//   generated at:  15.06.2007 11:45:47
//   generated by:  ALPHA-VISION/DataLink2Awl
//   project:       IMAC_L
//   user:          de2zehr0

FUNCTION "abvspu_T_API_FC" : VOID
TITLE =
VERSION : 0.1


VAR_TEMP
  rVal : REAL ;
  iVal : DINT ;
  wSts : INT ;
END_VAR
BEGIN
NETWORK
TITLE =API-Testfunktionen

      AUF   "abvspu_DB_DataLinkPLC";



      CALL "GetValueI" (
           obj                      := 1, // PointId = 011010, Station = PCU1
           iVal                     := #iVal);

      L     #iVal;
      T     DBD    2;


      CALL "GetValueI" (
           obj                      := 2505, // PointId = 011080, Station = PCU1
           iVal                     := #iVal);

      L     #iVal;
      T     DBD    6;


      CALL "GetValueI" (
           obj                      := 4, // PointId = 011160, Station = PCU1
           iVal                     := #iVal);

      L     #iVal;
      T     DBD    10;


      CALL "GetValueI" (
           obj                      := 5, // PointId = 011170, Station = PCU1
           iVal                     := #iVal);

      L     #iVal;
      T     DBD    14;


      CALL "GetValueI" (
           obj                      := 6, // PointId = 011180, Station = PCU1
           iVal                     := #iVal);

      L     #iVal;
      T     DBD    18;


      CALL "GetValueI" (
           obj                      := 8, // PointId = 011200, Station = PCU1
           iVal                     := #iVal);

      L     #iVal;
      T     DBD    22;


      CALL "GetValueI" (
           obj                      := 9, // PointId = 011210, Station = PCU1
           iVal                     := #iVal);

      L     #iVal;
      T     DBD    26;


      CALL "GetValueI" (
           obj                      := 2, // PointId = 011030, Station = PCU1
           iVal                     := #iVal);

      L     #iVal;
      T     DBD    30;


      CALL "GetValueI" (
           obj                      := 7, // PointId = 011190, Station = PCU1
           iVal                     := #iVal);

      L     #iVal;
      T     DBD    34;


      CALL "GetValueI" (
           obj                      := 10, // PointId = 011570, Station = PCU1
           iVal                     := #iVal);

      L     #iVal;
      T     DBD    38;


      CALL "GetValueR" (
           obj                      := 2503, // PointId = 011060, Station = PCU1
           rVal                     := #rVal);

      L     #rVal;
      T     DBD    42;


      CALL "GetValueR" (
           obj                      := 2505, // PointId = 011080, Station = PCU1
           rVal                     := #rVal);

      L     #rVal;
      T     DBD    46;


      CALL "GetValueR" (
           obj                      := 2506, // PointId = 011090, Station = PCU1
           rVal                     := #rVal);

      L     #rVal;
      T     DBD    50;


      CALL "GetValueR" (
           obj                      := 2508, // PointId = 011110, Station = PCU1
           rVal                     := #rVal);

      L     #rVal;
      T     DBD    54;


      CALL "GetValueR" (
           obj                      := 2510, // PointId = 011130, Station = PCU1
           rVal                     := #rVal);

      L     #rVal;
      T     DBD    58;


      CALL "GetValueR" (
           obj                      := 2500, // PointId = 011020, Station = PCU1
           rVal                     := #rVal);

      L     #rVal;
      T     DBD    62;


      CALL "GetValueR" (
           obj                      := 2501, // PointId = 011040, Station = PCU1
           rVal                     := #rVal);

      L     #rVal;
      T     DBD    66;


      CALL "GetValueR" (
           obj                      := 2502, // PointId = 011050, Station = PCU1
           rVal                     := #rVal);

      L     #rVal;
      T     DBD    70;


      CALL "GetValueR" (
           obj                      := 2504, // PointId = 011070, Station = PCU1
           rVal                     := #rVal);

      L     #rVal;
      T     DBD    74;


      CALL "GetValueR" (
           obj                      := 2507, // PointId = 011100, Station = PCU1
           rVal                     := #rVal);

      L     #rVal;
      T     DBD    78;


      CALL "GetValueR" (
           obj                      := 2509, // PointId = 011120, Station = PCU1
           rVal                     := #rVal);

      L     #rVal;
      T     DBD    82;


      CALL "GetValueR" (
           obj                      := 2511, // PointId = 011140, Station = PCU1
           rVal                     := #rVal);

      L     #rVal;
      T     DBD    86;


      CALL "GetValueR" (
           obj                      := 2512, // PointId = 011230, Station = PCU1
           rVal                     := #rVal);

      L     #rVal;
      T     DBD    90;


      CALL "GetValueR" (
           obj                      := 2513, // PointId = 011240, Station = PCU1
           rVal                     := #rVal);

      L     #rVal;
      T     DBD    94;


      CALL "GetValueR" (
           obj                      := 2514, // PointId = 011250, Station = PCU1
           rVal                     := #rVal);

      L     #rVal;
      T     DBD    98;


      CALL "GetValueR" (
           obj                      := 2515, // PointId = 011260, Station = PCU1
           rVal                     := #rVal);

      L     #rVal;
      T     DBD    102;


      CALL "GetValueR" (
           obj                      := 2516, // PointId = 011270, Station = PCU1
           rVal                     := #rVal);

      L     #rVal;
      T     DBD    106;


      CALL "GetValueR" (
           obj                      := 2517, // PointId = 011280, Station = PCU1
           rVal                     := #rVal);

      L     #rVal;
      T     DBD    110;


      CALL "GetValueR" (
           obj                      := 2518, // PointId = 011290, Station = PCU1
           rVal                     := #rVal);

      L     #rVal;
      T     DBD    114;


      CALL "GetValueR" (
           obj                      := 2519, // PointId = 011300, Station = PCU1
           rVal                     := #rVal);

      L     #rVal;
      T     DBD    118;


      CALL "GetValueR" (
           obj                      := 2520, // PointId = 011310, Station = PCU1
           rVal                     := #rVal);

      L     #rVal;
      T     DBD    122;


      CALL "GetValueR" (
           obj                      := 2521, // PointId = 011320, Station = PCU1
           rVal                     := #rVal);

      L     #rVal;
      T     DBD    126;


      CALL "GetValueR" (
           obj                      := 2522, // PointId = 011330, Station = PCU1
           rVal                     := #rVal);

      L     #rVal;
      T     DBD    130;


      CALL "GetValueR" (
           obj                      := 2523, // PointId = 011340, Station = PCU1
           rVal                     := #rVal);

      L     #rVal;
      T     DBD    134;


      CALL "GetValueR" (
           obj                      := 2524, // PointId = 011350, Station = PCU1
           rVal                     := #rVal);

      L     #rVal;
      T     DBD    138;


      CALL "GetValueR" (
           obj                      := 2525, // PointId = 011360, Station = PCU1
           rVal                     := #rVal);

      L     #rVal;
      T     DBD    142;


      CALL "GetValueR" (
           obj                      := 2526, // PointId = 011370, Station = PCU1
           rVal                     := #rVal);

      L     #rVal;
      T     DBD    146;


      CALL "GetValueR" (
           obj                      := 2527, // PointId = 011380, Station = PCU1
           rVal                     := #rVal);

      L     #rVal;
      T     DBD    150;


      CALL "GetValueR" (
           obj                      := 2544, // PointId = 011550, Station = PCU1
           rVal                     := #rVal);

      L     #rVal;
      T     DBD    154;


      CALL "GetValueR" (
           obj                      := 2545, // PointId = 011560, Station = PCU1
           rVal                     := #rVal);

      L     #rVal;
      T     DBD    158;


      CALL "GetValueI" (
           obj                      := 13, // PointId = 012010, Station = PCU1
           iVal                     := #iVal);

      L     #iVal;
      T     DBD    162;


      CALL "GetValueI" (
           obj                      := 2551, // PointId = 012080, Station = PCU1
           iVal                     := #iVal);

      L     #iVal;
      T     DBD    166;


      CALL "GetValueI" (
           obj                      := 16, // PointId = 012160, Station = PCU1
           iVal                     := #iVal);

      L     #iVal;
      T     DBD    170;


      CALL "GetValueI" (
           obj                      := 17, // PointId = 012170, Station = PCU1
           iVal                     := #iVal);

      L     #iVal;
      T     DBD    174;


      CALL "GetValueI" (
           obj                      := 18, // PointId = 012180, Station = PCU1
           iVal                     := #iVal);

      L     #iVal;
      T     DBD    178;


      CALL "GetValueI" (
           obj                      := 20, // PointId = 012200, Station = PCU1
           iVal                     := #iVal);

      L     #iVal;
      T     DBD    182;


      CALL "GetValueI" (
           obj                      := 21, // PointId = 012210, Station = PCU1
           iVal                     := #iVal);

      L     #iVal;
      T     DBD    186;


      CALL "GetValueI" (
           obj                      := 14, // PointId = 012030, Station = PCU1
           iVal                     := #iVal);

      L     #iVal;
      T     DBD    190;


      CALL "GetValueI" (
           obj                      := 19, // PointId = 012190, Station = PCU1
           iVal                     := #iVal);

      L     #iVal;
      T     DBD    194;


      CALL "GetValueI" (
           obj                      := 22, // PointId = 012570, Station = PCU1
           iVal                     := #iVal);

      L     #iVal;
      T     DBD    198;


      CALL "GetValueR" (
           obj                      := 2549, // PointId = 012060, Station = PCU1
           rVal                     := #rVal);

      L     #rVal;
      T     DBD    202;


      CALL "GetValueR" (
           obj                      := 2551, // PointId = 012080, Station = PCU1
           rVal                     := #rVal);

      L     #rVal;
      T     DBD    206;


      CALL "GetValueR" (
           obj                      := 2552, // PointId = 012090, Station = PCU1
           rVal                     := #rVal);

      L     #rVal;
      T     DBD    210;


      CALL "GetValueR" (
           obj                      := 2554, // PointId = 012110, Station = PCU1
           rVal                     := #rVal);

      L     #rVal;
      T     DBD    214;


      CALL "GetValueR" (
           obj                      := 2556, // PointId = 012130, Station = PCU1
           rVal                     := #rVal);

      L     #rVal;
      T     DBD    218;


      CALL "GetValueR" (
           obj                      := 2546, // PointId = 012020, Station = PCU1
           rVal                     := #rVal);

      L     #rVal;
      T     DBD    222;


      CALL "GetValueR" (
           obj                      := 2547, // PointId = 012040, Station = PCU1
           rVal                     := #rVal);

      L     #rVal;
      T     DBD    226;


      CALL "GetValueR" (
           obj                      := 2548, // PointId = 012050, Station = PCU1
           rVal                     := #rVal);

      L     #rVal;
      T     DBD    230;


      CALL "GetValueR" (
           obj                      := 2550, // PointId = 012070, Station = PCU1
           rVal                     := #rVal);

      L     #rVal;
      T     DBD    234;


      CALL "GetValueR" (
           obj                      := 2553, // PointId = 012100, Station = PCU1
           rVal                     := #rVal);

      L     #rVal;
      T     DBD    238;


      CALL "GetValueR" (
           obj                      := 2555, // PointId = 012120, Station = PCU1
           rVal                     := #rVal);

      L     #rVal;
      T     DBD    242;


      CALL "GetValueR" (
           obj                      := 2557, // PointId = 012140, Station = PCU1
           rVal                     := #rVal);

      L     #rVal;
      T     DBD    246;


      CALL "GetValueR" (
           obj                      := 2558, // PointId = 012230, Station = PCU1
           rVal                     := #rVal);

      L     #rVal;
      T     DBD    250;


      CALL "GetValueR" (
           obj                      := 2559, // PointId = 012240, Station = PCU1
           rVal                     := #rVal);

      L     #rVal;
      T     DBD    254;


      CALL "GetValueR" (
           obj                      := 2560, // PointId = 012250, Station = PCU1
           rVal                     := #rVal);

      L     #rVal;
      T     DBD    258;


      CALL "GetValueR" (
           obj                      := 2561, // PointId = 012260, Station = PCU1
           rVal                     := #rVal);

      L     #rVal;
      T     DBD    262;


      CALL "GetValueR" (
           obj                      := 2562, // PointId = 012270, Station = PCU1
           rVal                     := #rVal);

      L     #rVal;
      T     DBD    266;


      CALL "GetValueR" (
           obj                      := 2563, // PointId = 012280, Station = PCU1
           rVal                     := #rVal);

      L     #rVal;
      T     DBD    270;


      CALL "GetValueR" (
           obj                      := 2564, // PointId = 012290, Station = PCU1
           rVal                     := #rVal);

      L     #rVal;
      T     DBD    274;


      CALL "GetValueR" (
           obj                      := 2565, // PointId = 012300, Station = PCU1
           rVal                     := #rVal);

      L     #rVal;
      T     DBD    278;


      CALL "GetValueR" (
           obj                      := 2566, // PointId = 012310, Station = PCU1
           rVal                     := #rVal);

      L     #rVal;
      T     DBD    282;


      CALL "GetValueR" (
           obj                      := 2567, // PointId = 012320, Station = PCU1
           rVal                     := #rVal);

      L     #rVal;
      T     DBD    286;


      CALL "GetValueR" (
           obj                      := 2568, // PointId = 012330, Station = PCU1
           rVal                     := #rVal);

      L     #rVal;
      T     DBD    290;


      CALL "GetValueR" (
           obj                      := 2569, // PointId = 012340, Station = PCU1
           rVal                     := #rVal);

      L     #rVal;
      T     DBD    294;


      CALL "GetValueR" (
           obj                      := 2570, // PointId = 012350, Station = PCU1
           rVal                     := #rVal);

      L     #rVal;
      T     DBD    298;


      CALL "GetValueR" (
           obj                      := 2571, // PointId = 012360, Station = PCU1
           rVal                     := #rVal);

      L     #rVal;
      T     DBD    302;


      CALL "GetValueR" (
           obj                      := 2572, // PointId = 012370, Station = PCU1
           rVal                     := #rVal);

      L     #rVal;
      T     DBD    306;


      CALL "GetValueR" (
           obj                      := 2573, // PointId = 012380, Station = PCU1
           rVal                     := #rVal);

      L     #rVal;
      T     DBD    310;


      CALL "GetValueR" (
           obj                      := 2590, // PointId = 012550, Station = PCU1
           rVal                     := #rVal);

      L     #rVal;
      T     DBD    314;


      CALL "GetValueR" (
           obj                      := 2591, // PointId = 012560, Station = PCU1
           rVal                     := #rVal);

      L     #rVal;
      T     DBD    318;


      CALL "GetValueR" (
           obj                      := 2883, // PointId = 021010, Station = PCU1
           rVal                     := #rVal);

      L     #rVal;
      T     DBD    322;


      CALL "GetValueR" (
           obj                      := 2884, // PointId = 021020, Station = PCU1
           rVal                     := #rVal);

      L     #rVal;
      T     DBD    326;


      CALL "GetValueR" (
           obj                      := 2885, // PointId = 021030, Station = PCU1
           rVal                     := #rVal);

      L     #rVal;
      T     DBD    330;


      CALL "GetValueR" (
           obj                      := 2886, // PointId = 021040, Station = PCU1
           rVal                     := #rVal);

      L     #rVal;
      T     DBD    334;


      CALL "GetValueR" (
           obj                      := 2887, // PointId = 021051, Station = PCU1
           rVal                     := #rVal);

      L     #rVal;
      T     DBD    338;


      CALL "GetValueR" (
           obj                      := 2888, // PointId = 021060, Station = PCU1
           rVal                     := #rVal);

      L     #rVal;
      T     DBD    342;


      CALL "GetValueR" (
           obj                      := 2889, // PointId = 021070, Station = PCU1
           rVal                     := #rVal);

      L     #rVal;
      T     DBD    346;


      CALL "GetValueR" (
           obj                      := 2890, // PointId = 021080, Station = PCU1
           rVal                     := #rVal);

      L     #rVal;
      T     DBD    350;


      CALL "GetValueR" (
           obj                      := 2891, // PointId = 021090, Station = PCU1
           rVal                     := #rVal);

      L     #rVal;
      T     DBD    354;


      CALL "GetValueR" (
           obj                      := 2892, // PointId = 021120, Station = PCU1
           rVal                     := #rVal);

      L     #rVal;
      T     DBD    358;


      CALL "GetValueR" (
           obj                      := 2893, // PointId = 021130, Station = PCU1
           rVal                     := #rVal);

      L     #rVal;
      T     DBD    362;


      CALL "GetValueR" (
           obj                      := 2894, // PointId = 021140, Station = PCU1
           rVal                     := #rVal);

      L     #rVal;
      T     DBD    366;


      CALL "GetValueR" (
           obj                      := 2895, // PointId = 021150, Station = PCU1
           rVal                     := #rVal);

      L     #rVal;
      T     DBD    370;


      CALL "GetValueR" (
           obj                      := 2896, // PointId = 021160, Station = PCU1
           rVal                     := #rVal);

      L     #rVal;
      T     DBD    374;


      CALL "GetValueR" (
           obj                      := 2897, // PointId = 021170, Station = PCU1
           rVal                     := #rVal);

      L     #rVal;
      T     DBD    378;


      CALL "GetValueR" (
           obj                      := 2898, // PointId = 021180, Station = PCU1
           rVal                     := #rVal);

      L     #rVal;
      T     DBD    382;


      CALL "GetValueI" (
           obj                      := 140, // PointId = 021100, Station = PCU1
           iVal                     := #iVal);

      L     #iVal;
      T     DBD    386;


      CALL "GetValueI" (
           obj                      := 141, // PointId = 021110, Station = PCU1
           iVal                     := #iVal);

      L     #iVal;
      T     DBD    390;


      CALL "GetValueI" (
           obj                      := 142, // PointId = 021190, Station = PCU1
           iVal                     := #iVal);

      L     #iVal;
      T     DBD    394;


      CALL "GetValueI" (
           obj                      := 143, // PointId = 021200, Station = PCU1
           iVal                     := #iVal);

      L     #iVal;
      T     DBD    398;


      CALL "GetValueI" (
           obj                      := 144, // PointId = 021210, Station = PCU1
           iVal                     := #iVal);

      L     #iVal;
      T     DBD    402;


      CALL "GetValueI" (
           obj                      := 145, // PointId = 021240, Station = PCU1
           iVal                     := #iVal);

      L     #iVal;
      T     DBD    406;


      CALL "GetValueI" (
           obj                      := 146, // PointId = 021260, Station = PCU1
           iVal                     := #iVal);

      L     #iVal;
      T     DBD    410;


      CALL "GetValueI" (
           obj                      := 147, // PointId = 021270, Station = PCU1
           iVal                     := #iVal);

      L     #iVal;
      T     DBD    414;


      CALL "GetValueI" (
           obj                      := 148, // PointId = 021290, Station = PCU1
           iVal                     := #iVal);

      L     #iVal;
      T     DBD    418;


      CALL "GetValueI" (
           obj                      := 149, // PointId = 021310, Station = PCU1
           iVal                     := #iVal);

      L     #iVal;
      T     DBD    422;


      CALL "GetValueR" (
           obj                      := 2900, // PointId = 021300, Station = PCU1
           rVal                     := #rVal);

      L     #rVal;
      T     DBD    426;


      CALL "GetValueR" (
           obj                      := 2901, // PointId = 022010, Station = PCU1
           rVal                     := #rVal);

      L     #rVal;
      T     DBD    430;


      CALL "GetValueR" (
           obj                      := 2902, // PointId = 022020, Station = PCU1
           rVal                     := #rVal);

      L     #rVal;
      T     DBD    434;


      CALL "GetValueR" (
           obj                      := 2903, // PointId = 022030, Station = PCU1
           rVal                     := #rVal);

      L     #rVal;
      T     DBD    438;


      CALL "GetValueR" (
           obj                      := 2904, // PointId = 022040, Station = PCU1
           rVal                     := #rVal);

      L     #rVal;
      T     DBD    442;


      CALL "GetValueR" (
           obj                      := 2905, // PointId = 022051, Station = PCU1
           rVal                     := #rVal);

      L     #rVal;
      T     DBD    446;


      CALL "GetValueR" (
           obj                      := 2906, // PointId = 022060, Station = PCU1
           rVal                     := #rVal);

      L     #rVal;
      T     DBD    450;


      CALL "GetValueR" (
           obj                      := 2907, // PointId = 022070, Station = PCU1
           rVal                     := #rVal);

      L     #rVal;
      T     DBD    454;


      CALL "GetValueR" (
           obj                      := 2908, // PointId = 022080, Station = PCU1
           rVal                     := #rVal);

      L     #rVal;
      T     DBD    458;


      CALL "GetValueR" (
           obj                      := 2909, // PointId = 022090, Station = PCU1
           rVal                     := #rVal);

      L     #rVal;
      T     DBD    462;


      CALL "GetValueR" (
           obj                      := 2910, // PointId = 022120, Station = PCU1
           rVal                     := #rVal);

      L     #rVal;
      T     DBD    466;


      CALL "GetValueR" (
           obj                      := 2911, // PointId = 022130, Station = PCU1
           rVal                     := #rVal);

      L     #rVal;
      T     DBD    470;


      CALL "GetValueR" (
           obj                      := 2912, // PointId = 022140, Station = PCU1
           rVal                     := #rVal);

      L     #rVal;
      T     DBD    474;


      CALL "GetValueR" (
           obj                      := 2913, // PointId = 022150, Station = PCU1
           rVal                     := #rVal);

      L     #rVal;
      T     DBD    478;


      CALL "GetValueR" (
           obj                      := 2914, // PointId = 022160, Station = PCU1
           rVal                     := #rVal);

      L     #rVal;
      T     DBD    482;


      CALL "GetValueR" (
           obj                      := 2915, // PointId = 022170, Station = PCU1
           rVal                     := #rVal);

      L     #rVal;
      T     DBD    486;


      CALL "GetValueR" (
           obj                      := 2916, // PointId = 022180, Station = PCU1
           rVal                     := #rVal);

      L     #rVal;
      T     DBD    490;


      CALL "GetValueI" (
           obj                      := 152, // PointId = 022100, Station = PCU1
           iVal                     := #iVal);

      L     #iVal;
      T     DBD    494;


      CALL "GetValueI" (
           obj                      := 153, // PointId = 022110, Station = PCU1
           iVal                     := #iVal);

      L     #iVal;
      T     DBD    498;


      CALL "GetValueI" (
           obj                      := 154, // PointId = 022190, Station = PCU1
           iVal                     := #iVal);

      L     #iVal;
      T     DBD    502;


      CALL "GetValueI" (
           obj                      := 155, // PointId = 022200, Station = PCU1
           iVal                     := #iVal);

      L     #iVal;
      T     DBD    506;


      CALL "GetValueI" (
           obj                      := 156, // PointId = 022210, Station = PCU1
           iVal                     := #iVal);

      L     #iVal;
      T     DBD    510;


      CALL "GetValueI" (
           obj                      := 157, // PointId = 022240, Station = PCU1
           iVal                     := #iVal);

      L     #iVal;
      T     DBD    514;


      CALL "GetValueI" (
           obj                      := 158, // PointId = 022260, Station = PCU1
           iVal                     := #iVal);

      L     #iVal;
      T     DBD    518;


      CALL "GetValueI" (
           obj                      := 159, // PointId = 022270, Station = PCU1
           iVal                     := #iVal);

      L     #iVal;
      T     DBD    522;


      CALL "GetValueI" (
           obj                      := 160, // PointId = 022290, Station = PCU1
           iVal                     := #iVal);

      L     #iVal;
      T     DBD    526;


      CALL "GetValueI" (
           obj                      := 161, // PointId = 022310, Station = PCU1
           iVal                     := #iVal);

      L     #iVal;
      T     DBD    530;


      CALL "GetValueR" (
           obj                      := 2918, // PointId = 022300, Station = PCU1
           rVal                     := #rVal);

      L     #rVal;
      T     DBD    534;


      CALL "GetValueI" (
           obj                      := 25, // PointId = 013010, Station = PCU1
           iVal                     := #iVal);

      L     #iVal;
      T     DBD    538;


      CALL "GetValueI" (
           obj                      := 2597, // PointId = 013080, Station = PCU1
           iVal                     := #iVal);

      L     #iVal;
      T     DBD    542;


      CALL "GetValueI" (
           obj                      := 28, // PointId = 013160, Station = PCU1
           iVal                     := #iVal);

      L     #iVal;
      T     DBD    546;


      CALL "GetValueI" (
           obj                      := 29, // PointId = 013170, Station = PCU1
           iVal                     := #iVal);

      L     #iVal;
      T     DBD    550;


      CALL "GetValueI" (
           obj                      := 30, // PointId = 013180, Station = PCU1
           iVal                     := #iVal);

      L     #iVal;
      T     DBD    554;


      CALL "GetValueI" (
           obj                      := 32, // PointId = 013200, Station = PCU1
           iVal                     := #iVal);

      L     #iVal;
      T     DBD    558;


      CALL "GetValueI" (
           obj                      := 33, // PointId = 013210, Station = PCU1
           iVal                     := #iVal);

      L     #iVal;
      T     DBD    562;


      CALL "GetValueI" (
           obj                      := 26, // PointId = 013030, Station = PCU1
           iVal                     := #iVal);

      L     #iVal;
      T     DBD    566;


      CALL "GetValueI" (
           obj                      := 31, // PointId = 013190, Station = PCU1
           iVal                     := #iVal);

      L     #iVal;
      T     DBD    570;


      CALL "GetValueI" (
           obj                      := 34, // PointId = 013570, Station = PCU1
           iVal                     := #iVal);

      L     #iVal;
      T     DBD    574;


      CALL "GetValueR" (
           obj                      := 2595, // PointId = 013060, Station = PCU1
           rVal                     := #rVal);

      L     #rVal;
      T     DBD    578;


      CALL "GetValueR" (
           obj                      := 2597, // PointId = 013080, Station = PCU1
           rVal                     := #rVal);

      L     #rVal;
      T     DBD    582;


      CALL "GetValueR" (
           obj                      := 2598, // PointId = 013090, Station = PCU1
           rVal                     := #rVal);

      L     #rVal;
      T     DBD    586;


      CALL "GetValueR" (
           obj                      := 2600, // PointId = 013110, Station = PCU1
           rVal                     := #rVal);

      L     #rVal;
      T     DBD    590;


      CALL "GetValueR" (
           obj                      := 2602, // PointId = 013130, Station = PCU1
           rVal                     := #rVal);

      L     #rVal;
      T     DBD    594;


      CALL "GetValueR" (
           obj                      := 2592, // PointId = 013020, Station = PCU1
           rVal                     := #rVal);

      L     #rVal;
      T     DBD    598;


      CALL "GetValueR" (
           obj                      := 2593, // PointId = 013040, Station = PCU1
           rVal                     := #rVal);

      L     #rVal;
      T     DBD    602;


      CALL "GetValueR" (
           obj                      := 2594, // PointId = 013050, Station = PCU1
           rVal                     := #rVal);

      L     #rVal;
      T     DBD    606;


      CALL "GetValueR" (
           obj                      := 2596, // PointId = 013070, Station = PCU1
           rVal                     := #rVal);

      L     #rVal;
      T     DBD    610;


      CALL "GetValueR" (
           obj                      := 2599, // PointId = 013100, Station = PCU1
           rVal                     := #rVal);

      L     #rVal;
      T     DBD    614;


      CALL "GetValueR" (
           obj                      := 2601, // PointId = 013120, Station = PCU1
           rVal                     := #rVal);

      L     #rVal;
      T     DBD    618;


      CALL "GetValueR" (
           obj                      := 2603, // PointId = 013140, Station = PCU1
           rVal                     := #rVal);

      L     #rVal;
      T     DBD    622;


      CALL "GetValueR" (
           obj                      := 2604, // PointId = 013230, Station = PCU1
           rVal                     := #rVal);

      L     #rVal;
      T     DBD    626;


      CALL "GetValueR" (
           obj                      := 2605, // PointId = 013240, Station = PCU1
           rVal                     := #rVal);

      L     #rVal;
      T     DBD    630;


      CALL "GetValueR" (
           obj                      := 2606, // PointId = 013250, Station = PCU1
           rVal                     := #rVal);

      L     #rVal;
      T     DBD    634;


      CALL "GetValueR" (
           obj                      := 2607, // PointId = 013260, Station = PCU1
           rVal                     := #rVal);

      L     #rVal;
      T     DBD    638;


      CALL "GetValueR" (
           obj                      := 2608, // PointId = 013270, Station = PCU1
           rVal                     := #rVal);

      L     #rVal;
      T     DBD    642;


      CALL "GetValueR" (
           obj                      := 2609, // PointId = 013280, Station = PCU1
           rVal                     := #rVal);

      L     #rVal;
      T     DBD    646;


      CALL "GetValueR" (
           obj                      := 2610, // PointId = 013290, Station = PCU1
           rVal                     := #rVal);

      L     #rVal;
      T     DBD    650;


      CALL "GetValueR" (
           obj                      := 2611, // PointId = 013300, Station = PCU1
           rVal                     := #rVal);

      L     #rVal;
      T     DBD    654;


      CALL "GetValueR" (
           obj                      := 2612, // PointId = 013310, Station = PCU1
           rVal                     := #rVal);

      L     #rVal;
      T     DBD    658;


      CALL "GetValueR" (
           obj                      := 2613, // PointId = 013320, Station = PCU1
           rVal                     := #rVal);

      L     #rVal;
      T     DBD    662;


      CALL "GetValueR" (
           obj                      := 2614, // PointId = 013330, Station = PCU1
           rVal                     := #rVal);

      L     #rVal;
      T     DBD    666;


      CALL "GetValueR" (
           obj                      := 2615, // PointId = 013340, Station = PCU1
           rVal                     := #rVal);

      L     #rVal;
      T     DBD    670;


      CALL "GetValueR" (
           obj                      := 2616, // PointId = 013350, Station = PCU1
           rVal                     := #rVal);

      L     #rVal;
      T     DBD    674;


      CALL "GetValueR" (
           obj                      := 2617, // PointId = 013360, Station = PCU1
           rVal                     := #rVal);

      L     #rVal;
      T     DBD    678;


      CALL "GetValueR" (
           obj                      := 2618, // PointId = 013370, Station = PCU1
           rVal                     := #rVal);

      L     #rVal;
      T     DBD    682;


      CALL "GetValueR" (
           obj                      := 2619, // PointId = 013380, Station = PCU1
           rVal                     := #rVal);

      L     #rVal;
      T     DBD    686;


      CALL "GetValueR" (
           obj                      := 2636, // PointId = 013550, Station = PCU1
           rVal                     := #rVal);

      L     #rVal;
      T     DBD    690;


      CALL "GetValueR" (
           obj                      := 2637, // PointId = 013560, Station = PCU1
           rVal                     := #rVal);

      L     #rVal;
      T     DBD    694;


      CALL "GetValueI" (
           obj                      := 37, // PointId = 014010, Station = PCU1
           iVal                     := #iVal);

      L     #iVal;
      T     DBD    698;


      CALL "GetValueI" (
           obj                      := 2643, // PointId = 014080, Station = PCU1
           iVal                     := #iVal);

      L     #iVal;
      T     DBD    702;


      CALL "GetValueI" (
           obj                      := 40, // PointId = 014160, Station = PCU1
           iVal                     := #iVal);

      L     #iVal;
      T     DBD    706;


      CALL "GetValueI" (
           obj                      := 41, // PointId = 014170, Station = PCU1
           iVal                     := #iVal);

      L     #iVal;
      T     DBD    710;


      CALL "GetValueI" (
           obj                      := 42, // PointId = 014180, Station = PCU1
           iVal                     := #iVal);

      L     #iVal;
      T     DBD    714;


      CALL "GetValueI" (
           obj                      := 44, // PointId = 014200, Station = PCU1
           iVal                     := #iVal);

      L     #iVal;
      T     DBD    718;


      CALL "GetValueI" (
           obj                      := 45, // PointId = 014210, Station = PCU1
           iVal                     := #iVal);

      L     #iVal;
      T     DBD    722;


      CALL "GetValueI" (
           obj                      := 38, // PointId = 014030, Station = PCU1
           iVal                     := #iVal);

      L     #iVal;
      T     DBD    726;


      CALL "GetValueI" (
           obj                      := 43, // PointId = 014190, Station = PCU1
           iVal                     := #iVal);

      L     #iVal;
      T     DBD    730;


      CALL "GetValueI" (
           obj                      := 46, // PointId = 014570, Station = PCU1
           iVal                     := #iVal);

      L     #iVal;
      T     DBD    734;


      CALL "GetValueR" (
           obj                      := 2641, // PointId = 014060, Station = PCU1
           rVal                     := #rVal);

      L     #rVal;
      T     DBD    738;


      CALL "GetValueR" (
           obj                      := 2643, // PointId = 014080, Station = PCU1
           rVal                     := #rVal);

      L     #rVal;
      T     DBD    742;


      CALL "GetValueR" (
           obj                      := 2644, // PointId = 014090, Station = PCU1
           rVal                     := #rVal);

      L     #rVal;
      T     DBD    746;


      CALL "GetValueR" (
           obj                      := 2646, // PointId = 014110, Station = PCU1
           rVal                     := #rVal);

      L     #rVal;
      T     DBD    750;


      CALL "GetValueR" (
           obj                      := 2648, // PointId = 014130, Station = PCU1
           rVal                     := #rVal);

      L     #rVal;
      T     DBD    754;


      CALL "GetValueR" (
           obj                      := 2638, // PointId = 014020, Station = PCU1
           rVal                     := #rVal);

      L     #rVal;
      T     DBD    758;


      CALL "GetValueR" (
           obj                      := 2639, // PointId = 014040, Station = PCU1
           rVal                     := #rVal);

      L     #rVal;
      T     DBD    762;


      CALL "GetValueR" (
           obj                      := 2640, // PointId = 014050, Station = PCU1
           rVal                     := #rVal);

      L     #rVal;
      T     DBD    766;


      CALL "GetValueR" (
           obj                      := 2642, // PointId = 014070, Station = PCU1
           rVal                     := #rVal);

      L     #rVal;
      T     DBD    770;


      CALL "GetValueR" (
           obj                      := 2645, // PointId = 014100, Station = PCU1
           rVal                     := #rVal);

      L     #rVal;
      T     DBD    774;


      CALL "GetValueR" (
           obj                      := 2647, // PointId = 014120, Station = PCU1
           rVal                     := #rVal);

      L     #rVal;
      T     DBD    778;


      CALL "GetValueR" (
           obj                      := 2649, // PointId = 014140, Station = PCU1
           rVal                     := #rVal);

      L     #rVal;
      T     DBD    782;


      CALL "GetValueR" (
           obj                      := 2650, // PointId = 014230, Station = PCU1
           rVal                     := #rVal);

      L     #rVal;
      T     DBD    786;


      CALL "GetValueR" (
           obj                      := 2651, // PointId = 014240, Station = PCU1
           rVal                     := #rVal);

      L     #rVal;
      T     DBD    790;


      CALL "GetValueR" (
           obj                      := 2652, // PointId = 014250, Station = PCU1
           rVal                     := #rVal);

      L     #rVal;
      T     DBD    794;


      CALL "GetValueR" (
           obj                      := 2653, // PointId = 014260, Station = PCU1
           rVal                     := #rVal);

      L     #rVal;
      T     DBD    798;


      CALL "GetValueR" (
           obj                      := 2654, // PointId = 014270, Station = PCU1
           rVal                     := #rVal);

      L     #rVal;
      T     DBD    802;


      CALL "GetValueR" (
           obj                      := 2655, // PointId = 014280, Station = PCU1
           rVal                     := #rVal);

      L     #rVal;
      T     DBD    806;


      CALL "GetValueR" (
           obj                      := 2656, // PointId = 014290, Station = PCU1
           rVal                     := #rVal);

      L     #rVal;
      T     DBD    810;


      CALL "GetValueR" (
           obj                      := 2657, // PointId = 014300, Station = PCU1
           rVal                     := #rVal);

      L     #rVal;
      T     DBD    814;


      CALL "GetValueR" (
           obj                      := 2658, // PointId = 014310, Station = PCU1
           rVal                     := #rVal);

      L     #rVal;
      T     DBD    818;


      CALL "GetValueR" (
           obj                      := 2659, // PointId = 014320, Station = PCU1
           rVal                     := #rVal);

      L     #rVal;
      T     DBD    822;


      CALL "GetValueR" (
           obj                      := 2660, // PointId = 014330, Station = PCU1
           rVal                     := #rVal);

      L     #rVal;
      T     DBD    826;


      CALL "GetValueR" (
           obj                      := 2661, // PointId = 014340, Station = PCU1
           rVal                     := #rVal);

      L     #rVal;
      T     DBD    830;


      CALL "GetValueR" (
           obj                      := 2662, // PointId = 014350, Station = PCU1
           rVal                     := #rVal);

      L     #rVal;
      T     DBD    834;


      CALL "GetValueR" (
           obj                      := 2663, // PointId = 014360, Station = PCU1
           rVal                     := #rVal);

      L     #rVal;
      T     DBD    838;


      CALL "GetValueR" (
           obj                      := 2664, // PointId = 014370, Station = PCU1
           rVal                     := #rVal);

      L     #rVal;
      T     DBD    842;


      CALL "GetValueR" (
           obj                      := 2665, // PointId = 014380, Station = PCU1
           rVal                     := #rVal);

      L     #rVal;
      T     DBD    846;


      CALL "GetValueR" (
           obj                      := 2682, // PointId = 014550, Station = PCU1
           rVal                     := #rVal);

      L     #rVal;
      T     DBD    850;


      CALL "GetValueR" (
           obj                      := 2683, // PointId = 014560, Station = PCU1
           rVal                     := #rVal);

      L     #rVal;
      T     DBD    854;


      CALL "GetValueR" (
           obj                      := 2919, // PointId = 023010, Station = PCU1
           rVal                     := #rVal);

      L     #rVal;
      T     DBD    858;


      CALL "GetValueR" (
           obj                      := 2920, // PointId = 023020, Station = PCU1
           rVal                     := #rVal);

      L     #rVal;
      T     DBD    862;


      CALL "GetValueR" (
           obj                      := 2921, // PointId = 023030, Station = PCU1
           rVal                     := #rVal);

      L     #rVal;
      T     DBD    866;


      CALL "GetValueR" (
           obj                      := 2922, // PointId = 023040, Station = PCU1
           rVal                     := #rVal);

      L     #rVal;
      T     DBD    870;


      CALL "GetValueR" (
           obj                      := 2923, // PointId = 023051, Station = PCU1
           rVal                     := #rVal);

      L     #rVal;
      T     DBD    874;


      CALL "GetValueR" (
           obj                      := 2924, // PointId = 023060, Station = PCU1
           rVal                     := #rVal);

      L     #rVal;
      T     DBD    878;


      CALL "GetValueR" (
           obj                      := 2925, // PointId = 023070, Station = PCU1
           rVal                     := #rVal);

      L     #rVal;
      T     DBD    882;


      CALL "GetValueR" (
           obj                      := 2926, // PointId = 023080, Station = PCU1
           rVal                     := #rVal);

      L     #rVal;
      T     DBD    886;


      CALL "GetValueR" (
           obj                      := 2927, // PointId = 023090, Station = PCU1
           rVal                     := #rVal);

      L     #rVal;
      T     DBD    890;


      CALL "GetValueR" (
           obj                      := 2928, // PointId = 023120, Station = PCU1
           rVal                     := #rVal);

      L     #rVal;
      T     DBD    894;


      CALL "GetValueR" (
           obj                      := 2929, // PointId = 023130, Station = PCU1
           rVal                     := #rVal);

      L     #rVal;
      T     DBD    898;


      CALL "GetValueR" (
           obj                      := 2930, // PointId = 023140, Station = PCU1
           rVal                     := #rVal);

      L     #rVal;
      T     DBD    902;


      CALL "GetValueR" (
           obj                      := 2931, // PointId = 023150, Station = PCU1
           rVal                     := #rVal);

      L     #rVal;
      T     DBD    906;


      CALL "GetValueR" (
           obj                      := 2932, // PointId = 023160, Station = PCU1
           rVal                     := #rVal);

      L     #rVal;
      T     DBD    910;


      CALL "GetValueR" (
           obj                      := 2933, // PointId = 023170, Station = PCU1
           rVal                     := #rVal);

      L     #rVal;
      T     DBD    914;


      CALL "GetValueR" (
           obj                      := 2934, // PointId = 023180, Station = PCU1
           rVal                     := #rVal);

      L     #rVal;
      T     DBD    918;


      CALL "GetValueI" (
           obj                      := 164, // PointId = 023100, Station = PCU1
           iVal                     := #iVal);

      L     #iVal;
      T     DBD    922;


      CALL "GetValueI" (
           obj                      := 165, // PointId = 023110, Station = PCU1
           iVal                     := #iVal);

      L     #iVal;
      T     DBD    926;


      CALL "GetValueI" (
           obj                      := 166, // PointId = 023190, Station = PCU1
           iVal                     := #iVal);

      L     #iVal;
      T     DBD    930;


      CALL "GetValueI" (
           obj                      := 167, // PointId = 023200, Station = PCU1
           iVal                     := #iVal);

      L     #iVal;
      T     DBD    934;


      CALL "GetValueI" (
           obj                      := 168, // PointId = 023210, Station = PCU1
           iVal                     := #iVal);

      L     #iVal;
      T     DBD    938;


      CALL "GetValueI" (
           obj                      := 169, // PointId = 023240, Station = PCU1
           iVal                     := #iVal);

      L     #iVal;
      T     DBD    942;


      CALL "GetValueI" (
           obj                      := 170, // PointId = 023260, Station = PCU1
           iVal                     := #iVal);

      L     #iVal;
      T     DBD    946;


      CALL "GetValueI" (
           obj                      := 171, // PointId = 023270, Station = PCU1
           iVal                     := #iVal);

      L     #iVal;
      T     DBD    950;


      CALL "GetValueI" (
           obj                      := 172, // PointId = 023290, Station = PCU1
           iVal                     := #iVal);

      L     #iVal;
      T     DBD    954;


      CALL "GetValueI" (
           obj                      := 173, // PointId = 023310, Station = PCU1
           iVal                     := #iVal);

      L     #iVal;
      T     DBD    958;


      CALL "GetValueR" (
           obj                      := 2936, // PointId = 023300, Station = PCU1
           rVal                     := #rVal);

      L     #rVal;
      T     DBD    962;


      CALL "GetValueR" (
           obj                      := 2937, // PointId = 024010, Station = PCU1
           rVal                     := #rVal);

      L     #rVal;
      T     DBD    966;


      CALL "GetValueR" (
           obj                      := 2938, // PointId = 024020, Station = PCU1
           rVal                     := #rVal);

      L     #rVal;
      T     DBD    970;


      CALL "GetValueR" (
           obj                      := 2939, // PointId = 024030, Station = PCU1
           rVal                     := #rVal);

      L     #rVal;
      T     DBD    974;


      CALL "GetValueR" (
           obj                      := 2940, // PointId = 024040, Station = PCU1
           rVal                     := #rVal);

      L     #rVal;
      T     DBD    978;


      CALL "GetValueR" (
           obj                      := 2941, // PointId = 024051, Station = PCU1
           rVal                     := #rVal);

      L     #rVal;
      T     DBD    982;


      CALL "GetValueR" (
           obj                      := 2942, // PointId = 024060, Station = PCU1
           rVal                     := #rVal);

      L     #rVal;
      T     DBD    986;


      CALL "GetValueR" (
           obj                      := 2943, // PointId = 024070, Station = PCU1
           rVal                     := #rVal);

      L     #rVal;
      T     DBD    990;


      CALL "GetValueR" (
           obj                      := 2944, // PointId = 024080, Station = PCU1
           rVal                     := #rVal);

      L     #rVal;
      T     DBD    994;


      CALL "GetValueR" (
           obj                      := 2945, // PointId = 024090, Station = PCU1
           rVal                     := #rVal);

      L     #rVal;
      T     DBD    998;


      CALL "GetValueR" (
           obj                      := 2946, // PointId = 024120, Station = PCU1
           rVal                     := #rVal);

      L     #rVal;
      T     DBD    1002;


      CALL "GetValueR" (
           obj                      := 2947, // PointId = 024130, Station = PCU1
           rVal                     := #rVal);

      L     #rVal;
      T     DBD    1006;


      CALL "GetValueR" (
           obj                      := 2948, // PointId = 024140, Station = PCU1
           rVal                     := #rVal);

      L     #rVal;
      T     DBD    1010;


      CALL "GetValueR" (
           obj                      := 2949, // PointId = 024150, Station = PCU1
           rVal                     := #rVal);

      L     #rVal;
      T     DBD    1014;


      CALL "GetValueR" (
           obj                      := 2950, // PointId = 024160, Station = PCU1
           rVal                     := #rVal);

      L     #rVal;
      T     DBD    1018;


      CALL "GetValueR" (
           obj                      := 2951, // PointId = 024170, Station = PCU1
           rVal                     := #rVal);

      L     #rVal;
      T     DBD    1022;


      CALL "GetValueR" (
           obj                      := 2952, // PointId = 024180, Station = PCU1
           rVal                     := #rVal);

      L     #rVal;
      T     DBD    1026;


      CALL "GetValueI" (
           obj                      := 176, // PointId = 024100, Station = PCU1
           iVal                     := #iVal);

      L     #iVal;
      T     DBD    1030;


      CALL "GetValueI" (
           obj                      := 177, // PointId = 024110, Station = PCU1
           iVal                     := #iVal);

      L     #iVal;
      T     DBD    1034;


      CALL "GetValueI" (
           obj                      := 178, // PointId = 024190, Station = PCU1
           iVal                     := #iVal);

      L     #iVal;
      T     DBD    1038;


      CALL "GetValueI" (
           obj                      := 179, // PointId = 024200, Station = PCU1
           iVal                     := #iVal);

      L     #iVal;
      T     DBD    1042;


      CALL "GetValueI" (
           obj                      := 180, // PointId = 024210, Station = PCU1
           iVal                     := #iVal);

      L     #iVal;
      T     DBD    1046;


      CALL "GetValueI" (
           obj                      := 181, // PointId = 024240, Station = PCU1
           iVal                     := #iVal);

      L     #iVal;
      T     DBD    1050;


      CALL "GetValueI" (
           obj                      := 182, // PointId = 024260, Station = PCU1
           iVal                     := #iVal);

      L     #iVal;
      T     DBD    1054;


      CALL "GetValueI" (
           obj                      := 183, // PointId = 024270, Station = PCU1
           iVal                     := #iVal);

      L     #iVal;
      T     DBD    1058;


      CALL "GetValueI" (
           obj                      := 184, // PointId = 024290, Station = PCU1
           iVal                     := #iVal);

      L     #iVal;
      T     DBD    1062;


      CALL "GetValueI" (
           obj                      := 185, // PointId = 024310, Station = PCU1
           iVal                     := #iVal);

      L     #iVal;
      T     DBD    1066;


      CALL "GetValueR" (
           obj                      := 2954, // PointId = 024300, Station = PCU1
           rVal                     := #rVal);

      L     #rVal;
      T     DBD    1070;


      CALL "GetValueI" (
           obj                      := 49, // PointId = 015010, Station = PCU1
           iVal                     := #iVal);

      L     #iVal;
      T     DBD    1074;


      CALL "GetValueI" (
           obj                      := 2689, // PointId = 015080, Station = PCU1
           iVal                     := #iVal);

      L     #iVal;
      T     DBD    1078;


      CALL "GetValueI" (
           obj                      := 52, // PointId = 015160, Station = PCU1
           iVal                     := #iVal);

      L     #iVal;
      T     DBD    1082;


      CALL "GetValueI" (
           obj                      := 53, // PointId = 015170, Station = PCU1
           iVal                     := #iVal);

      L     #iVal;
      T     DBD    1086;


      CALL "GetValueI" (
           obj                      := 54, // PointId = 015180, Station = PCU1
           iVal                     := #iVal);

      L     #iVal;
      T     DBD    1090;


      CALL "GetValueI" (
           obj                      := 56, // PointId = 015200, Station = PCU1
           iVal                     := #iVal);

      L     #iVal;
      T     DBD    1094;


      CALL "GetValueI" (
           obj                      := 57, // PointId = 015210, Station = PCU1
           iVal                     := #iVal);

      L     #iVal;
      T     DBD    1098;


      CALL "GetValueI" (
           obj                      := 50, // PointId = 015030, Station = PCU1
           iVal                     := #iVal);

      L     #iVal;
      T     DBD    1102;


      CALL "GetValueI" (
           obj                      := 55, // PointId = 015190, Station = PCU1
           iVal                     := #iVal);

      L     #iVal;
      T     DBD    1106;


      CALL "GetValueI" (
           obj                      := 58, // PointId = 015570, Station = PCU1
           iVal                     := #iVal);

      L     #iVal;
      T     DBD    1110;


      CALL "GetValueR" (
           obj                      := 2687, // PointId = 015060, Station = PCU1
           rVal                     := #rVal);

      L     #rVal;
      T     DBD    1114;


      CALL "GetValueR" (
           obj                      := 2689, // PointId = 015080, Station = PCU1
           rVal                     := #rVal);

      L     #rVal;
      T     DBD    1118;


      CALL "GetValueR" (
           obj                      := 2690, // PointId = 015090, Station = PCU1
           rVal                     := #rVal);

      L     #rVal;
      T     DBD    1122;


      CALL "GetValueR" (
           obj                      := 2692, // PointId = 015110, Station = PCU1
           rVal                     := #rVal);

      L     #rVal;
      T     DBD    1126;


      CALL "GetValueR" (
           obj                      := 2694, // PointId = 015130, Station = PCU1
           rVal                     := #rVal);

      L     #rVal;
      T     DBD    1130;


      CALL "GetValueR" (
           obj                      := 2684, // PointId = 015020, Station = PCU1
           rVal                     := #rVal);

      L     #rVal;
      T     DBD    1134;


      CALL "GetValueR" (
           obj                      := 2685, // PointId = 015040, Station = PCU1
           rVal                     := #rVal);

      L     #rVal;
      T     DBD    1138;


      CALL "GetValueR" (
           obj                      := 2686, // PointId = 015050, Station = PCU1
           rVal                     := #rVal);

      L     #rVal;
      T     DBD    1142;


      CALL "GetValueR" (
           obj                      := 2688, // PointId = 015070, Station = PCU1
           rVal                     := #rVal);

      L     #rVal;
      T     DBD    1146;


      CALL "GetValueR" (
           obj                      := 2691, // PointId = 015100, Station = PCU1
           rVal                     := #rVal);

      L     #rVal;
      T     DBD    1150;


      CALL "GetValueR" (
           obj                      := 2693, // PointId = 015120, Station = PCU1
           rVal                     := #rVal);

      L     #rVal;
      T     DBD    1154;


      CALL "GetValueR" (
           obj                      := 2695, // PointId = 015140, Station = PCU1
           rVal                     := #rVal);

      L     #rVal;
      T     DBD    1158;


      CALL "GetValueR" (
           obj                      := 2696, // PointId = 015230, Station = PCU1
           rVal                     := #rVal);

      L     #rVal;
      T     DBD    1162;


      CALL "GetValueR" (
           obj                      := 2697, // PointId = 015240, Station = PCU1
           rVal                     := #rVal);

      L     #rVal;
      T     DBD    1166;


      CALL "GetValueR" (
           obj                      := 2698, // PointId = 015250, Station = PCU1
           rVal                     := #rVal);

      L     #rVal;
      T     DBD    1170;


      CALL "GetValueR" (
           obj                      := 2699, // PointId = 015260, Station = PCU1
           rVal                     := #rVal);

      L     #rVal;
      T     DBD    1174;


      CALL "GetValueR" (
           obj                      := 2700, // PointId = 015270, Station = PCU1
           rVal                     := #rVal);

      L     #rVal;
      T     DBD    1178;


      CALL "GetValueR" (
           obj                      := 2701, // PointId = 015280, Station = PCU1
           rVal                     := #rVal);

      L     #rVal;
      T     DBD    1182;


      CALL "GetValueR" (
           obj                      := 2702, // PointId = 015290, Station = PCU1
           rVal                     := #rVal);

      L     #rVal;
      T     DBD    1186;


      CALL "GetValueR" (
           obj                      := 2703, // PointId = 015300, Station = PCU1
           rVal                     := #rVal);

      L     #rVal;
      T     DBD    1190;


      CALL "GetValueR" (
           obj                      := 2704, // PointId = 015310, Station = PCU1
           rVal                     := #rVal);

      L     #rVal;
      T     DBD    1194;


      CALL "GetValueR" (
           obj                      := 2705, // PointId = 015320, Station = PCU1
           rVal                     := #rVal);

      L     #rVal;
      T     DBD    1198;


      CALL "GetValueR" (
           obj                      := 2706, // PointId = 015330, Station = PCU1
           rVal                     := #rVal);

      L     #rVal;
      T     DBD    1202;


      CALL "GetValueR" (
           obj                      := 2707, // PointId = 015340, Station = PCU1
           rVal                     := #rVal);

      L     #rVal;
      T     DBD    1206;


      CALL "GetValueR" (
           obj                      := 2708, // PointId = 015350, Station = PCU1
           rVal                     := #rVal);

      L     #rVal;
      T     DBD    1210;


      CALL "GetValueR" (
           obj                      := 2709, // PointId = 015360, Station = PCU1
           rVal                     := #rVal);

      L     #rVal;
      T     DBD    1214;


      CALL "GetValueR" (
           obj                      := 2710, // PointId = 015370, Station = PCU1
           rVal                     := #rVal);

      L     #rVal;
      T     DBD    1218;


      CALL "GetValueR" (
           obj                      := 2711, // PointId = 015380, Station = PCU1
           rVal                     := #rVal);

      L     #rVal;
      T     DBD    1222;


      CALL "GetValueR" (
           obj                      := 2728, // PointId = 015550, Station = PCU1
           rVal                     := #rVal);

      L     #rVal;
      T     DBD    1226;


      CALL "GetValueR" (
           obj                      := 2729, // PointId = 015560, Station = PCU1
           rVal                     := #rVal);

      L     #rVal;
      T     DBD    1230;


      CALL "GetValueI" (
           obj                      := 61, // PointId = 016010, Station = PCU1
           iVal                     := #iVal);

      L     #iVal;
      T     DBD    1234;


      CALL "GetValueI" (
           obj                      := 2735, // PointId = 016080, Station = PCU1
           iVal                     := #iVal);

      L     #iVal;
      T     DBD    1238;


      CALL "GetValueI" (
           obj                      := 64, // PointId = 016160, Station = PCU1
           iVal                     := #iVal);

      L     #iVal;
      T     DBD    1242;


      CALL "GetValueI" (
           obj                      := 65, // PointId = 016170, Station = PCU1
           iVal                     := #iVal);

      L     #iVal;
      T     DBD    1246;


      CALL "GetValueI" (
           obj                      := 66, // PointId = 016180, Station = PCU1
           iVal                     := #iVal);

      L     #iVal;
      T     DBD    1250;


      CALL "GetValueI" (
           obj                      := 68, // PointId = 016200, Station = PCU1
           iVal                     := #iVal);

      L     #iVal;
      T     DBD    1254;


      CALL "GetValueI" (
           obj                      := 69, // PointId = 016210, Station = PCU1
           iVal                     := #iVal);

      L     #iVal;
      T     DBD    1258;


      CALL "GetValueI" (
           obj                      := 62, // PointId = 016030, Station = PCU1
           iVal                     := #iVal);

      L     #iVal;
      T     DBD    1262;


      CALL "GetValueI" (
           obj                      := 67, // PointId = 016190, Station = PCU1
           iVal                     := #iVal);

      L     #iVal;
      T     DBD    1266;


      CALL "GetValueI" (
           obj                      := 70, // PointId = 016570, Station = PCU1
           iVal                     := #iVal);

      L     #iVal;
      T     DBD    1270;


      CALL "GetValueR" (
           obj                      := 2733, // PointId = 016060, Station = PCU1
           rVal                     := #rVal);

      L     #rVal;
      T     DBD    1274;


      CALL "GetValueR" (
           obj                      := 2735, // PointId = 016080, Station = PCU1
           rVal                     := #rVal);

      L     #rVal;
      T     DBD    1278;


      CALL "GetValueR" (
           obj                      := 2736, // PointId = 016090, Station = PCU1
           rVal                     := #rVal);

      L     #rVal;
      T     DBD    1282;


      CALL "GetValueR" (
           obj                      := 2738, // PointId = 016110, Station = PCU1
           rVal                     := #rVal);

      L     #rVal;
      T     DBD    1286;


      CALL "GetValueR" (
           obj                      := 2740, // PointId = 016130, Station = PCU1
           rVal                     := #rVal);

      L     #rVal;
      T     DBD    1290;


      CALL "GetValueR" (
           obj                      := 2730, // PointId = 016020, Station = PCU1
           rVal                     := #rVal);

      L     #rVal;
      T     DBD    1294;


      CALL "GetValueR" (
           obj                      := 2731, // PointId = 016040, Station = PCU1
           rVal                     := #rVal);

      L     #rVal;
      T     DBD    1298;


      CALL "GetValueR" (
           obj                      := 2732, // PointId = 016050, Station = PCU1
           rVal                     := #rVal);

      L     #rVal;
      T     DBD    1302;


      CALL "GetValueR" (
           obj                      := 2734, // PointId = 016070, Station = PCU1
           rVal                     := #rVal);

      L     #rVal;
      T     DBD    1306;


      CALL "GetValueR" (
           obj                      := 2737, // PointId = 016100, Station = PCU1
           rVal                     := #rVal);

      L     #rVal;
      T     DBD    1310;


      CALL "GetValueR" (
           obj                      := 2739, // PointId = 016120, Station = PCU1
           rVal                     := #rVal);

      L     #rVal;
      T     DBD    1314;


      CALL "GetValueR" (
           obj                      := 2741, // PointId = 016140, Station = PCU1
           rVal                     := #rVal);

      L     #rVal;
      T     DBD    1318;


      CALL "GetValueR" (
           obj                      := 2742, // PointId = 016230, Station = PCU1
           rVal                     := #rVal);

      L     #rVal;
      T     DBD    1322;


      CALL "GetValueR" (
           obj                      := 2743, // PointId = 016240, Station = PCU1
           rVal                     := #rVal);

      L     #rVal;
      T     DBD    1326;


      CALL "GetValueR" (
           obj                      := 2744, // PointId = 016250, Station = PCU1
           rVal                     := #rVal);

      L     #rVal;
      T     DBD    1330;


      CALL "GetValueR" (
           obj                      := 2745, // PointId = 016260, Station = PCU1
           rVal                     := #rVal);

      L     #rVal;
      T     DBD    1334;


      CALL "GetValueR" (
           obj                      := 2746, // PointId = 016270, Station = PCU1
           rVal                     := #rVal);

      L     #rVal;
      T     DBD    1338;


      CALL "GetValueR" (
           obj                      := 2747, // PointId = 016280, Station = PCU1
           rVal                     := #rVal);

      L     #rVal;
      T     DBD    1342;


      CALL "GetValueR" (
           obj                      := 2748, // PointId = 016290, Station = PCU1
           rVal                     := #rVal);

      L     #rVal;
      T     DBD    1346;


      CALL "GetValueR" (
           obj                      := 2749, // PointId = 016300, Station = PCU1
           rVal                     := #rVal);

      L     #rVal;
      T     DBD    1350;


      CALL "GetValueR" (
           obj                      := 2750, // PointId = 016310, Station = PCU1
           rVal                     := #rVal);

      L     #rVal;
      T     DBD    1354;


      CALL "GetValueR" (
           obj                      := 2751, // PointId = 016320, Station = PCU1
           rVal                     := #rVal);

      L     #rVal;
      T     DBD    1358;


      CALL "GetValueR" (
           obj                      := 2752, // PointId = 016330, Station = PCU1
           rVal                     := #rVal);

      L     #rVal;
      T     DBD    1362;


      CALL "GetValueR" (
           obj                      := 2753, // PointId = 016340, Station = PCU1
           rVal                     := #rVal);

      L     #rVal;
      T     DBD    1366;


      CALL "GetValueR" (
           obj                      := 2754, // PointId = 016350, Station = PCU1
           rVal                     := #rVal);

      L     #rVal;
      T     DBD    1370;


      CALL "GetValueR" (
           obj                      := 2755, // PointId = 016360, Station = PCU1
           rVal                     := #rVal);

      L     #rVal;
      T     DBD    1374;


      CALL "GetValueR" (
           obj                      := 2756, // PointId = 016370, Station = PCU1
           rVal                     := #rVal);

      L     #rVal;
      T     DBD    1378;


      CALL "GetValueR" (
           obj                      := 2757, // PointId = 016380, Station = PCU1
           rVal                     := #rVal);

      L     #rVal;
      T     DBD    1382;


      CALL "GetValueR" (
           obj                      := 2774, // PointId = 016550, Station = PCU1
           rVal                     := #rVal);

      L     #rVal;
      T     DBD    1386;


      CALL "GetValueR" (
           obj                      := 2775, // PointId = 016560, Station = PCU1
           rVal                     := #rVal);

      L     #rVal;
      T     DBD    1390;


      CALL "GetValueR" (
           obj                      := 2955, // PointId = 025010, Station = PCU1
           rVal                     := #rVal);

      L     #rVal;
      T     DBD    1394;


      CALL "GetValueR" (
           obj                      := 2956, // PointId = 025020, Station = PCU1
           rVal                     := #rVal);

      L     #rVal;
      T     DBD    1398;


      CALL "GetValueR" (
           obj                      := 2957, // PointId = 025030, Station = PCU1
           rVal                     := #rVal);

      L     #rVal;
      T     DBD    1402;


      CALL "GetValueR" (
           obj                      := 2958, // PointId = 025040, Station = PCU1
           rVal                     := #rVal);

      L     #rVal;
      T     DBD    1406;


      CALL "GetValueR" (
           obj                      := 2959, // PointId = 025051, Station = PCU1
           rVal                     := #rVal);

      L     #rVal;
      T     DBD    1410;


      CALL "GetValueR" (
           obj                      := 2960, // PointId = 025060, Station = PCU1
           rVal                     := #rVal);

      L     #rVal;
      T     DBD    1414;


      CALL "GetValueR" (
           obj                      := 2961, // PointId = 025070, Station = PCU1
           rVal                     := #rVal);

      L     #rVal;
      T     DBD    1418;


      CALL "GetValueR" (
           obj                      := 2962, // PointId = 025080, Station = PCU1
           rVal                     := #rVal);

      L     #rVal;
      T     DBD    1422;


      CALL "GetValueR" (
           obj                      := 2963, // PointId = 025090, Station = PCU1
           rVal                     := #rVal);

      L     #rVal;
      T     DBD    1426;


      CALL "GetValueR" (
           obj                      := 2964, // PointId = 025120, Station = PCU1
           rVal                     := #rVal);

      L     #rVal;
      T     DBD    1430;


      CALL "GetValueR" (
           obj                      := 2965, // PointId = 025130, Station = PCU1
           rVal                     := #rVal);

      L     #rVal;
      T     DBD    1434;


      CALL "GetValueR" (
           obj                      := 2966, // PointId = 025140, Station = PCU1
           rVal                     := #rVal);

      L     #rVal;
      T     DBD    1438;


      CALL "GetValueR" (
           obj                      := 2967, // PointId = 025150, Station = PCU1
           rVal                     := #rVal);

      L     #rVal;
      T     DBD    1442;


      CALL "GetValueR" (
           obj                      := 2968, // PointId = 025160, Station = PCU1
           rVal                     := #rVal);

      L     #rVal;
      T     DBD    1446;


      CALL "GetValueR" (
           obj                      := 2969, // PointId = 025170, Station = PCU1
           rVal                     := #rVal);

      L     #rVal;
      T     DBD    1450;


      CALL "GetValueR" (
           obj                      := 2970, // PointId = 025180, Station = PCU1
           rVal                     := #rVal);

      L     #rVal;
      T     DBD    1454;


      CALL "GetValueI" (
           obj                      := 188, // PointId = 025100, Station = PCU1
           iVal                     := #iVal);

      L     #iVal;
      T     DBD    1458;


      CALL "GetValueI" (
           obj                      := 189, // PointId = 025110, Station = PCU1
           iVal                     := #iVal);

      L     #iVal;
      T     DBD    1462;


      CALL "GetValueI" (
           obj                      := 190, // PointId = 025190, Station = PCU1
           iVal                     := #iVal);

      L     #iVal;
      T     DBD    1466;


      CALL "GetValueI" (
           obj                      := 191, // PointId = 025200, Station = PCU1
           iVal                     := #iVal);

      L     #iVal;
      T     DBD    1470;


      CALL "GetValueI" (
           obj                      := 192, // PointId = 025210, Station = PCU1
           iVal                     := #iVal);

      L     #iVal;
      T     DBD    1474;


      CALL "GetValueI" (
           obj                      := 193, // PointId = 025240, Station = PCU1
           iVal                     := #iVal);

      L     #iVal;
      T     DBD    1478;


      CALL "GetValueI" (
           obj                      := 194, // PointId = 025260, Station = PCU1
           iVal                     := #iVal);

      L     #iVal;
      T     DBD    1482;


      CALL "GetValueI" (
           obj                      := 195, // PointId = 025270, Station = PCU1
           iVal                     := #iVal);

      L     #iVal;
      T     DBD    1486;


      CALL "GetValueI" (
           obj                      := 196, // PointId = 025290, Station = PCU1
           iVal                     := #iVal);

      L     #iVal;
      T     DBD    1490;


      CALL "GetValueI" (
           obj                      := 197, // PointId = 025310, Station = PCU1
           iVal                     := #iVal);

      L     #iVal;
      T     DBD    1494;


      CALL "GetValueR" (
           obj                      := 2972, // PointId = 025300, Station = PCU1
           rVal                     := #rVal);

      L     #rVal;
      T     DBD    1498;


      CALL "GetValueR" (
           obj                      := 2973, // PointId = 026010, Station = PCU1
           rVal                     := #rVal);

      L     #rVal;
      T     DBD    1502;


      CALL "GetValueR" (
           obj                      := 2974, // PointId = 026020, Station = PCU1
           rVal                     := #rVal);

      L     #rVal;
      T     DBD    1506;


      CALL "GetValueR" (
           obj                      := 2975, // PointId = 026030, Station = PCU1
           rVal                     := #rVal);

      L     #rVal;
      T     DBD    1510;


      CALL "GetValueR" (
           obj                      := 2976, // PointId = 026040, Station = PCU1
           rVal                     := #rVal);

      L     #rVal;
      T     DBD    1514;


      CALL "GetValueR" (
           obj                      := 2977, // PointId = 026051, Station = PCU1
           rVal                     := #rVal);

      L     #rVal;
      T     DBD    1518;


      CALL "GetValueR" (
           obj                      := 2978, // PointId = 026060, Station = PCU1
           rVal                     := #rVal);

      L     #rVal;
      T     DBD    1522;


      CALL "GetValueR" (
           obj                      := 2979, // PointId = 026070, Station = PCU1
           rVal                     := #rVal);

      L     #rVal;
      T     DBD    1526;


      CALL "GetValueR" (
           obj                      := 2980, // PointId = 026080, Station = PCU1
           rVal                     := #rVal);

      L     #rVal;
      T     DBD    1530;


      CALL "GetValueR" (
           obj                      := 2981, // PointId = 026090, Station = PCU1
           rVal                     := #rVal);

      L     #rVal;
      T     DBD    1534;


      CALL "GetValueR" (
           obj                      := 2982, // PointId = 026120, Station = PCU1
           rVal                     := #rVal);

      L     #rVal;
      T     DBD    1538;


      CALL "GetValueR" (
           obj                      := 2983, // PointId = 026130, Station = PCU1
           rVal                     := #rVal);

      L     #rVal;
      T     DBD    1542;


      CALL "GetValueR" (
           obj                      := 2984, // PointId = 026140, Station = PCU1
           rVal                     := #rVal);

      L     #rVal;
      T     DBD    1546;


      CALL "GetValueR" (
           obj                      := 2985, // PointId = 026150, Station = PCU1
           rVal                     := #rVal);

      L     #rVal;
      T     DBD    1550;


      CALL "GetValueR" (
           obj                      := 2986, // PointId = 026160, Station = PCU1
           rVal                     := #rVal);

      L     #rVal;
      T     DBD    1554;


      CALL "GetValueR" (
           obj                      := 2987, // PointId = 026170, Station = PCU1
           rVal                     := #rVal);

      L     #rVal;
      T     DBD    1558;


      CALL "GetValueR" (
           obj                      := 2988, // PointId = 026180, Station = PCU1
           rVal                     := #rVal);

      L     #rVal;
      T     DBD    1562;


      CALL "GetValueI" (
           obj                      := 200, // PointId = 026100, Station = PCU1
           iVal                     := #iVal);

      L     #iVal;
      T     DBD    1566;


      CALL "GetValueI" (
           obj                      := 201, // PointId = 026110, Station = PCU1
           iVal                     := #iVal);

      L     #iVal;
      T     DBD    1570;


      CALL "GetValueI" (
           obj                      := 202, // PointId = 026190, Station = PCU1
           iVal                     := #iVal);

      L     #iVal;
      T     DBD    1574;


      CALL "GetValueI" (
           obj                      := 203, // PointId = 026200, Station = PCU1
           iVal                     := #iVal);

      L     #iVal;
      T     DBD    1578;


      CALL "GetValueI" (
           obj                      := 204, // PointId = 026210, Station = PCU1
           iVal                     := #iVal);

      L     #iVal;
      T     DBD    1582;


      CALL "GetValueI" (
           obj                      := 205, // PointId = 026240, Station = PCU1
           iVal                     := #iVal);

      L     #iVal;
      T     DBD    1586;


      CALL "GetValueI" (
           obj                      := 206, // PointId = 026260, Station = PCU1
           iVal                     := #iVal);

      L     #iVal;
      T     DBD    1590;


      CALL "GetValueI" (
           obj                      := 207, // PointId = 026270, Station = PCU1
           iVal                     := #iVal);

      L     #iVal;
      T     DBD    1594;


      CALL "GetValueI" (
           obj                      := 208, // PointId = 026290, Station = PCU1
           iVal                     := #iVal);

      L     #iVal;
      T     DBD    1598;


      CALL "GetValueI" (
           obj                      := 209, // PointId = 026310, Station = PCU1
           iVal                     := #iVal);

      L     #iVal;
      T     DBD    1602;


      CALL "GetValueR" (
           obj                      := 2990, // PointId = 026300, Station = PCU1
           rVal                     := #rVal);

      L     #rVal;
      T     DBD    1606;


      CALL "GetValueI" (
           obj                      := 82, // PointId = 017110, Station = PCU1
           iVal                     := #iVal);

      L     #iVal;
      T     DBD    1610;


      CALL "GetValueI" (
           obj                      := 73, // PointId = 017010, Station = PCU1
           iVal                     := #iVal);

      L     #iVal;
      T     DBD    1614;


      CALL "GetValueI" (
           obj                      := 78, // PointId = 017070, Station = PCU1
           iVal                     := #iVal);

      L     #iVal;
      T     DBD    1618;


      CALL "GetValueI" (
           obj                      := 79, // PointId = 017080, Station = PCU1
           iVal                     := #iVal);

      L     #iVal;
      T     DBD    1622;


      CALL "GetValueI" (
           obj                      := 80, // PointId = 017090, Station = PCU1
           iVal                     := #iVal);

      L     #iVal;
      T     DBD    1626;


      CALL "GetValueI" (
           obj                      := 82, // PointId = 017110, Station = PCU1
           iVal                     := #iVal);

      L     #iVal;
      T     DBD    1630;


      CALL "GetValueI" (
           obj                      := 74, // PointId = 017020, Station = PCU1
           iVal                     := #iVal);

      L     #iVal;
      T     DBD    1634;


      CALL "GetValueI" (
           obj                      := 75, // PointId = 017030, Station = PCU1
           iVal                     := #iVal);

      L     #iVal;
      T     DBD    1638;


      CALL "GetValueI" (
           obj                      := 77, // PointId = 017060, Station = PCU1
           iVal                     := #iVal);

      L     #iVal;
      T     DBD    1642;


      CALL "GetValueI" (
           obj                      := 81, // PointId = 017100, Station = PCU1
           iVal                     := #iVal);

      L     #iVal;
      T     DBD    1646;


      CALL "GetValueI" (
           obj                      := 82, // PointId = 017110, Station = PCU1
           iVal                     := #iVal);

      L     #iVal;
      T     DBD    1650;


      CALL "GetValueI" (
           obj                      := 82, // PointId = 017110, Station = PCU1
           iVal                     := #iVal);

      L     #iVal;
      T     DBD    1654;


      CALL "GetValueI" (
           obj                      := 82, // PointId = 017110, Station = PCU1
           iVal                     := #iVal);

      L     #iVal;
      T     DBD    1658;


      CALL "GetValueI" (
           obj                      := 76, // PointId = 017050, Station = PCU1
           iVal                     := #iVal);

      L     #iVal;
      T     DBD    1662;


      CALL "GetValueI" (
           obj                      := 83, // PointId = 017490, Station = PCU1
           iVal                     := #iVal);

      L     #iVal;
      T     DBD    1666;


      CALL "GetValueR" (
           obj                      := 2776, // PointId = 017150, Station = PCU1
           rVal                     := #rVal);

      L     #rVal;
      T     DBD    1670;


      CALL "GetValueR" (
           obj                      := 2777, // PointId = 017160, Station = PCU1
           rVal                     := #rVal);

      L     #rVal;
      T     DBD    1674;


      CALL "GetValueR" (
           obj                      := 2778, // PointId = 017170, Station = PCU1
           rVal                     := #rVal);

      L     #rVal;
      T     DBD    1678;


      CALL "GetValueR" (
           obj                      := 2779, // PointId = 017180, Station = PCU1
           rVal                     := #rVal);

      L     #rVal;
      T     DBD    1682;


      CALL "GetValueR" (
           obj                      := 2780, // PointId = 017190, Station = PCU1
           rVal                     := #rVal);

      L     #rVal;
      T     DBD    1686;


      CALL "GetValueR" (
           obj                      := 2781, // PointId = 017200, Station = PCU1
           rVal                     := #rVal);

      L     #rVal;
      T     DBD    1690;


      CALL "GetValueR" (
           obj                      := 2782, // PointId = 017210, Station = PCU1
           rVal                     := #rVal);

      L     #rVal;
      T     DBD    1694;


      CALL "GetValueR" (
           obj                      := 2783, // PointId = 017220, Station = PCU1
           rVal                     := #rVal);

      L     #rVal;
      T     DBD    1698;


      CALL "GetValueR" (
           obj                      := 2784, // PointId = 017230, Station = PCU1
           rVal                     := #rVal);

      L     #rVal;
      T     DBD    1702;


      CALL "GetValueR" (
           obj                      := 2785, // PointId = 017240, Station = PCU1
           rVal                     := #rVal);

      L     #rVal;
      T     DBD    1706;


      CALL "GetValueR" (
           obj                      := 2786, // PointId = 017250, Station = PCU1
           rVal                     := #rVal);

      L     #rVal;
      T     DBD    1710;


      CALL "GetValueR" (
           obj                      := 2787, // PointId = 017260, Station = PCU1
           rVal                     := #rVal);

      L     #rVal;
      T     DBD    1714;


      CALL "GetValueR" (
           obj                      := 2788, // PointId = 017270, Station = PCU1
           rVal                     := #rVal);

      L     #rVal;
      T     DBD    1718;


      CALL "GetValueR" (
           obj                      := 2789, // PointId = 017280, Station = PCU1
           rVal                     := #rVal);

      L     #rVal;
      T     DBD    1722;


      CALL "GetValueR" (
           obj                      := 2790, // PointId = 017290, Station = PCU1
           rVal                     := #rVal);

      L     #rVal;
      T     DBD    1726;


      CALL "GetValueR" (
           obj                      := 2791, // PointId = 017300, Station = PCU1
           rVal                     := #rVal);

      L     #rVal;
      T     DBD    1730;


      CALL "GetValueR" (
           obj                      := 2808, // PointId = 017470, Station = PCU1
           rVal                     := #rVal);

      L     #rVal;
      T     DBD    1734;


      CALL "GetValueR" (
           obj                      := 2808, // PointId = 017470, Station = PCU1
           rVal                     := #rVal);

      L     #rVal;
      T     DBD    1738;


      CALL "GetValueI" (
           obj                      := 96, // PointId = 018110, Station = PCU1
           iVal                     := #iVal);

      L     #iVal;
      T     DBD    1742;


      CALL "GetValueI" (
           obj                      := 87, // PointId = 018010, Station = PCU1
           iVal                     := #iVal);

      L     #iVal;
      T     DBD    1746;


      CALL "GetValueI" (
           obj                      := 92, // PointId = 018070, Station = PCU1
           iVal                     := #iVal);

      L     #iVal;
      T     DBD    1750;


      CALL "GetValueI" (
           obj                      := 93, // PointId = 018080, Station = PCU1
           iVal                     := #iVal);

      L     #iVal;
      T     DBD    1754;


      CALL "GetValueI" (
           obj                      := 94, // PointId = 018090, Station = PCU1
           iVal                     := #iVal);

      L     #iVal;
      T     DBD    1758;


      CALL "GetValueI" (
           obj                      := 96, // PointId = 018110, Station = PCU1
           iVal                     := #iVal);

      L     #iVal;
      T     DBD    1762;


      CALL "GetValueI" (
           obj                      := 88, // PointId = 018020, Station = PCU1
           iVal                     := #iVal);

      L     #iVal;
      T     DBD    1766;


      CALL "GetValueI" (
           obj                      := 89, // PointId = 018030, Station = PCU1
           iVal                     := #iVal);

      L     #iVal;
      T     DBD    1770;


      CALL "GetValueI" (
           obj                      := 91, // PointId = 018060, Station = PCU1
           iVal                     := #iVal);

      L     #iVal;
      T     DBD    1774;


      CALL "GetValueI" (
           obj                      := 95, // PointId = 018100, Station = PCU1
           iVal                     := #iVal);

      L     #iVal;
      T     DBD    1778;


      CALL "GetValueI" (
           obj                      := 96, // PointId = 018110, Station = PCU1
           iVal                     := #iVal);

      L     #iVal;
      T     DBD    1782;


      CALL "GetValueI" (
           obj                      := 96, // PointId = 018110, Station = PCU1
           iVal                     := #iVal);

      L     #iVal;
      T     DBD    1786;


      CALL "GetValueI" (
           obj                      := 96, // PointId = 018110, Station = PCU1
           iVal                     := #iVal);

      L     #iVal;
      T     DBD    1790;


      CALL "GetValueI" (
           obj                      := 90, // PointId = 018050, Station = PCU1
           iVal                     := #iVal);

      L     #iVal;
      T     DBD    1794;


      CALL "GetValueI" (
           obj                      := 97, // PointId = 018490, Station = PCU1
           iVal                     := #iVal);

      L     #iVal;
      T     DBD    1798;


      CALL "GetValueR" (
           obj                      := 2809, // PointId = 018150, Station = PCU1
           rVal                     := #rVal);

      L     #rVal;
      T     DBD    1802;


      CALL "GetValueR" (
           obj                      := 2810, // PointId = 018160, Station = PCU1
           rVal                     := #rVal);

      L     #rVal;
      T     DBD    1806;


      CALL "GetValueR" (
           obj                      := 2811, // PointId = 018170, Station = PCU1
           rVal                     := #rVal);

      L     #rVal;
      T     DBD    1810;


      CALL "GetValueR" (
           obj                      := 2812, // PointId = 018180, Station = PCU1
           rVal                     := #rVal);

      L     #rVal;
      T     DBD    1814;


      CALL "GetValueR" (
           obj                      := 2813, // PointId = 018190, Station = PCU1
           rVal                     := #rVal);

      L     #rVal;
      T     DBD    1818;


      CALL "GetValueR" (
           obj                      := 2814, // PointId = 018200, Station = PCU1
           rVal                     := #rVal);

      L     #rVal;
      T     DBD    1822;


      CALL "GetValueR" (
           obj                      := 2815, // PointId = 018210, Station = PCU1
           rVal                     := #rVal);

      L     #rVal;
      T     DBD    1826;


      CALL "GetValueR" (
           obj                      := 2816, // PointId = 018220, Station = PCU1
           rVal                     := #rVal);

      L     #rVal;
      T     DBD    1830;


      CALL "GetValueR" (
           obj                      := 2817, // PointId = 018230, Station = PCU1
           rVal                     := #rVal);

      L     #rVal;
      T     DBD    1834;


      CALL "GetValueR" (
           obj                      := 2818, // PointId = 018240, Station = PCU1
           rVal                     := #rVal);

      L     #rVal;
      T     DBD    1838;


      CALL "GetValueR" (
           obj                      := 2819, // PointId = 018250, Station = PCU1
           rVal                     := #rVal);

      L     #rVal;
      T     DBD    1842;


      CALL "GetValueR" (
           obj                      := 2820, // PointId = 018260, Station = PCU1
           rVal                     := #rVal);

      L     #rVal;
      T     DBD    1846;


      CALL "GetValueR" (
           obj                      := 2821, // PointId = 018270, Station = PCU1
           rVal                     := #rVal);

      L     #rVal;
      T     DBD    1850;


      CALL "GetValueR" (
           obj                      := 2822, // PointId = 018280, Station = PCU1
           rVal                     := #rVal);

      L     #rVal;
      T     DBD    1854;


      CALL "GetValueR" (
           obj                      := 2823, // PointId = 018290, Station = PCU1
           rVal                     := #rVal);

      L     #rVal;
      T     DBD    1858;


      CALL "GetValueR" (
           obj                      := 2824, // PointId = 018300, Station = PCU1
           rVal                     := #rVal);

      L     #rVal;
      T     DBD    1862;


      CALL "GetValueR" (
           obj                      := 2841, // PointId = 018470, Station = PCU1
           rVal                     := #rVal);

      L     #rVal;
      T     DBD    1866;


      CALL "GetValueR" (
           obj                      := 2841, // PointId = 018470, Station = PCU1
           rVal                     := #rVal);

      L     #rVal;
      T     DBD    1870;


      CALL "GetValueR" (
           obj                      := 2991, // PointId = 027010, Station = PCU1
           rVal                     := #rVal);

      L     #rVal;
      T     DBD    1874;


      CALL "GetValueR" (
           obj                      := 2992, // PointId = 027020, Station = PCU1
           rVal                     := #rVal);

      L     #rVal;
      T     DBD    1878;


      CALL "GetValueR" (
           obj                      := 2993, // PointId = 027030, Station = PCU1
           rVal                     := #rVal);

      L     #rVal;
      T     DBD    1882;


      CALL "GetValueR" (
           obj                      := 2994, // PointId = 027040, Station = PCU1
           rVal                     := #rVal);

      L     #rVal;
      T     DBD    1886;


      CALL "GetValueR" (
           obj                      := 2995, // PointId = 027051, Station = PCU1
           rVal                     := #rVal);

      L     #rVal;
      T     DBD    1890;


      CALL "GetValueR" (
           obj                      := 2996, // PointId = 027060, Station = PCU1
           rVal                     := #rVal);

      L     #rVal;
      T     DBD    1894;


      CALL "GetValueR" (
           obj                      := 2997, // PointId = 027070, Station = PCU1
           rVal                     := #rVal);

      L     #rVal;
      T     DBD    1898;


      CALL "GetValueR" (
           obj                      := 2998, // PointId = 027080, Station = PCU1
           rVal                     := #rVal);

      L     #rVal;
      T     DBD    1902;


      CALL "GetValueR" (
           obj                      := 2999, // PointId = 027090, Station = PCU1
           rVal                     := #rVal);

      L     #rVal;
      T     DBD    1906;


      CALL "GetValueR" (
           obj                      := 3000, // PointId = 027120, Station = PCU1
           rVal                     := #rVal);

      L     #rVal;
      T     DBD    1910;


      CALL "GetValueR" (
           obj                      := 3001, // PointId = 027130, Station = PCU1
           rVal                     := #rVal);

      L     #rVal;
      T     DBD    1914;


      CALL "GetValueR" (
           obj                      := 3002, // PointId = 027140, Station = PCU1
           rVal                     := #rVal);

      L     #rVal;
      T     DBD    1918;


      CALL "GetValueR" (
           obj                      := 3003, // PointId = 027150, Station = PCU1
           rVal                     := #rVal);

      L     #rVal;
      T     DBD    1922;


      CALL "GetValueR" (
           obj                      := 3004, // PointId = 027160, Station = PCU1
           rVal                     := #rVal);

      L     #rVal;
      T     DBD    1926;


      CALL "GetValueR" (
           obj                      := 3004, // PointId = 027160, Station = PCU1
           rVal                     := #rVal);

      L     #rVal;
      T     DBD    1930;


      CALL "GetValueR" (
           obj                      := 3004, // PointId = 027160, Station = PCU1
           rVal                     := #rVal);

      L     #rVal;
      T     DBD    1934;


      CALL "GetValueI" (
           obj                      := 212, // PointId = 027100, Station = PCU1
           iVal                     := #iVal);

      L     #iVal;
      T     DBD    1938;


      CALL "GetValueI" (
           obj                      := 213, // PointId = 027110, Station = PCU1
           iVal                     := #iVal);

      L     #iVal;
      T     DBD    1942;


      CALL "GetValueI" (
           obj                      := 214, // PointId = 027190, Station = PCU1
           iVal                     := #iVal);

      L     #iVal;
      T     DBD    1946;


      CALL "GetValueI" (
           obj                      := 215, // PointId = 027200, Station = PCU1
           iVal                     := #iVal);

      L     #iVal;
      T     DBD    1950;


      CALL "GetValueI" (
           obj                      := 216, // PointId = 027210, Station = PCU1
           iVal                     := #iVal);

      L     #iVal;
      T     DBD    1954;


      CALL "GetValueI" (
           obj                      := 217, // PointId = 027240, Station = PCU1
           iVal                     := #iVal);

      L     #iVal;
      T     DBD    1958;


      CALL "GetValueI" (
           obj                      := 218, // PointId = 027260, Station = PCU1
           iVal                     := #iVal);

      L     #iVal;
      T     DBD    1962;


      CALL "GetValueI" (
           obj                      := 219, // PointId = 027270, Station = PCU1
           iVal                     := #iVal);

      L     #iVal;
      T     DBD    1966;


      CALL "GetValueI" (
           obj                      := 220, // PointId = 027290, Station = PCU1
           iVal                     := #iVal);

      L     #iVal;
      T     DBD    1970;


      CALL "GetValueI" (
           obj                      := 220, // PointId = 027290, Station = PCU1
           iVal                     := #iVal);

      L     #iVal;
      T     DBD    1974;


      CALL "GetValueR" (
           obj                      := 3006, // PointId = 027300, Station = PCU1
           rVal                     := #rVal);

      L     #rVal;
      T     DBD    1978;


      CALL "GetValueR" (
           obj                      := 3007, // PointId = 028010, Station = PCU1
           rVal                     := #rVal);

      L     #rVal;
      T     DBD    1982;


      CALL "GetValueR" (
           obj                      := 3008, // PointId = 028020, Station = PCU1
           rVal                     := #rVal);

      L     #rVal;
      T     DBD    1986;


      CALL "GetValueR" (
           obj                      := 3009, // PointId = 028030, Station = PCU1
           rVal                     := #rVal);

      L     #rVal;
      T     DBD    1990;


      CALL "GetValueR" (
           obj                      := 3010, // PointId = 028040, Station = PCU1
           rVal                     := #rVal);

      L     #rVal;
      T     DBD    1994;


      CALL "GetValueR" (
           obj                      := 3011, // PointId = 028051, Station = PCU1
           rVal                     := #rVal);

      L     #rVal;
      T     DBD    1998;


      CALL "GetValueR" (
           obj                      := 3012, // PointId = 028060, Station = PCU1
           rVal                     := #rVal);

      L     #rVal;
      T     DBD    2002;


      CALL "GetValueR" (
           obj                      := 3013, // PointId = 028070, Station = PCU1
           rVal                     := #rVal);

      L     #rVal;
      T     DBD    2006;


      CALL "GetValueR" (
           obj                      := 3014, // PointId = 028080, Station = PCU1
           rVal                     := #rVal);

      L     #rVal;
      T     DBD    2010;


      CALL "GetValueR" (
           obj                      := 3015, // PointId = 028090, Station = PCU1
           rVal                     := #rVal);

      L     #rVal;
      T     DBD    2014;


      CALL "GetValueR" (
           obj                      := 3016, // PointId = 028120, Station = PCU1
           rVal                     := #rVal);

      L     #rVal;
      T     DBD    2018;


      CALL "GetValueR" (
           obj                      := 3017, // PointId = 028130, Station = PCU1
           rVal                     := #rVal);

      L     #rVal;
      T     DBD    2022;


      CALL "GetValueR" (
           obj                      := 3018, // PointId = 028140, Station = PCU1
           rVal                     := #rVal);

      L     #rVal;
      T     DBD    2026;


      CALL "GetValueR" (
           obj                      := 3019, // PointId = 028150, Station = PCU1
           rVal                     := #rVal);

      L     #rVal;
      T     DBD    2030;


      CALL "GetValueR" (
           obj                      := 3020, // PointId = 028160, Station = PCU1
           rVal                     := #rVal);

      L     #rVal;
      T     DBD    2034;


      CALL "GetValueR" (
           obj                      := 3020, // PointId = 028160, Station = PCU1
           rVal                     := #rVal);

      L     #rVal;
      T     DBD    2038;


      CALL "GetValueR" (
           obj                      := 3020, // PointId = 028160, Station = PCU1
           rVal                     := #rVal);

      L     #rVal;
      T     DBD    2042;


      CALL "GetValueI" (
           obj                      := 223, // PointId = 028100, Station = PCU1
           iVal                     := #iVal);

      L     #iVal;
      T     DBD    2046;


      CALL "GetValueI" (
           obj                      := 224, // PointId = 028110, Station = PCU1
           iVal                     := #iVal);

      L     #iVal;
      T     DBD    2050;


      CALL "GetValueI" (
           obj                      := 225, // PointId = 028190, Station = PCU1
           iVal                     := #iVal);

      L     #iVal;
      T     DBD    2054;


      CALL "GetValueI" (
           obj                      := 226, // PointId = 028200, Station = PCU1
           iVal                     := #iVal);

      L     #iVal;
      T     DBD    2058;


      CALL "GetValueI" (
           obj                      := 227, // PointId = 028210, Station = PCU1
           iVal                     := #iVal);

      L     #iVal;
      T     DBD    2062;


      CALL "GetValueI" (
           obj                      := 228, // PointId = 028240, Station = PCU1
           iVal                     := #iVal);

      L     #iVal;
      T     DBD    2066;


      CALL "GetValueI" (
           obj                      := 229, // PointId = 028260, Station = PCU1
           iVal                     := #iVal);

      L     #iVal;
      T     DBD    2070;


      CALL "GetValueI" (
           obj                      := 230, // PointId = 028270, Station = PCU1
           iVal                     := #iVal);

      L     #iVal;
      T     DBD    2074;


      CALL "GetValueI" (
           obj                      := 231, // PointId = 028290, Station = PCU1
           iVal                     := #iVal);

      L     #iVal;
      T     DBD    2078;


      CALL "GetValueI" (
           obj                      := 231, // PointId = 028290, Station = PCU1
           iVal                     := #iVal);

      L     #iVal;
      T     DBD    2082;


      CALL "GetValueR" (
           obj                      := 3022, // PointId = 028300, Station = PCU1
           rVal                     := #rVal);

      L     #rVal;
      T     DBD    2086;


      CALL "GetValueI" (
           obj                      := 110, // PointId = 019110, Station = PCU1
           iVal                     := #iVal);

      L     #iVal;
      T     DBD    2090;


      CALL "GetValueI" (
           obj                      := 101, // PointId = 019010, Station = PCU1
           iVal                     := #iVal);

      L     #iVal;
      T     DBD    2094;


      CALL "GetValueI" (
           obj                      := 106, // PointId = 019070, Station = PCU1
           iVal                     := #iVal);

      L     #iVal;
      T     DBD    2098;


      CALL "GetValueI" (
           obj                      := 107, // PointId = 019080, Station = PCU1
           iVal                     := #iVal);

      L     #iVal;
      T     DBD    2102;


      CALL "GetValueI" (
           obj                      := 108, // PointId = 019090, Station = PCU1
           iVal                     := #iVal);

      L     #iVal;
      T     DBD    2106;


      CALL "GetValueI" (
           obj                      := 110, // PointId = 019110, Station = PCU1
           iVal                     := #iVal);

      L     #iVal;
      T     DBD    2110;


      CALL "GetValueI" (
           obj                      := 102, // PointId = 019020, Station = PCU1
           iVal                     := #iVal);

      L     #iVal;
      T     DBD    2114;


      CALL "GetValueI" (
           obj                      := 103, // PointId = 019030, Station = PCU1
           iVal                     := #iVal);

      L     #iVal;
      T     DBD    2118;


      CALL "GetValueI" (
           obj                      := 105, // PointId = 019060, Station = PCU1
           iVal                     := #iVal);

      L     #iVal;
      T     DBD    2122;


      CALL "GetValueI" (
           obj                      := 109, // PointId = 019100, Station = PCU1
           iVal                     := #iVal);

      L     #iVal;
      T     DBD    2126;


      CALL "GetValueI" (
           obj                      := 110, // PointId = 019110, Station = PCU1
           iVal                     := #iVal);

      L     #iVal;
      T     DBD    2130;


      CALL "GetValueI" (
           obj                      := 110, // PointId = 019110, Station = PCU1
           iVal                     := #iVal);

      L     #iVal;
      T     DBD    2134;


      CALL "GetValueI" (
           obj                      := 110, // PointId = 019110, Station = PCU1
           iVal                     := #iVal);

      L     #iVal;
      T     DBD    2138;


      CALL "GetValueI" (
           obj                      := 104, // PointId = 019050, Station = PCU1
           iVal                     := #iVal);

      L     #iVal;
      T     DBD    2142;


      CALL "GetValueI" (
           obj                      := 111, // PointId = 019490, Station = PCU1
           iVal                     := #iVal);

      L     #iVal;
      T     DBD    2146;


      CALL "GetValueR" (
           obj                      := 2842, // PointId = 019150, Station = PCU1
           rVal                     := #rVal);

      L     #rVal;
      T     DBD    2150;


      CALL "GetValueR" (
           obj                      := 2843, // PointId = 019160, Station = PCU1
           rVal                     := #rVal);

      L     #rVal;
      T     DBD    2154;


      CALL "GetValueR" (
           obj                      := 2844, // PointId = 019170, Station = PCU1
           rVal                     := #rVal);

      L     #rVal;
      T     DBD    2158;


      CALL "GetValueR" (
           obj                      := 2845, // PointId = 019180, Station = PCU1
           rVal                     := #rVal);

      L     #rVal;
      T     DBD    2162;


      CALL "GetValueR" (
           obj                      := 2846, // PointId = 019190, Station = PCU1
           rVal                     := #rVal);

      L     #rVal;
      T     DBD    2166;


      CALL "GetValueR" (
           obj                      := 2847, // PointId = 019200, Station = PCU1
           rVal                     := #rVal);

      L     #rVal;
      T     DBD    2170;


      CALL "GetValueR" (
           obj                      := 2848, // PointId = 019210, Station = PCU1
           rVal                     := #rVal);

      L     #rVal;
      T     DBD    2174;


      CALL "GetValueR" (
           obj                      := 2849, // PointId = 019220, Station = PCU1
           rVal                     := #rVal);

      L     #rVal;
      T     DBD    2178;


      CALL "GetValueR" (
           obj                      := 2850, // PointId = 019230, Station = PCU1
           rVal                     := #rVal);

      L     #rVal;
      T     DBD    2182;


      CALL "GetValueR" (
           obj                      := 2851, // PointId = 019240, Station = PCU1
           rVal                     := #rVal);

      L     #rVal;
      T     DBD    2186;


      CALL "GetValueR" (
           obj                      := 2852, // PointId = 019250, Station = PCU1
           rVal                     := #rVal);

      L     #rVal;
      T     DBD    2190;


      CALL "GetValueR" (
           obj                      := 2853, // PointId = 019260, Station = PCU1
           rVal                     := #rVal);

      L     #rVal;
      T     DBD    2194;


      CALL "GetValueR" (
           obj                      := 2854, // PointId = 019270, Station = PCU1
           rVal                     := #rVal);

      L     #rVal;
      T     DBD    2198;


      CALL "GetValueR" (
           obj                      := 2855, // PointId = 019280, Station = PCU1
           rVal                     := #rVal);

      L     #rVal;
      T     DBD    2202;


      CALL "GetValueR" (
           obj                      := 2856, // PointId = 019290, Station = PCU1
           rVal                     := #rVal);

      L     #rVal;
      T     DBD    2206;


      CALL "GetValueR" (
           obj                      := 2857, // PointId = 019300, Station = PCU1
           rVal                     := #rVal);

      L     #rVal;
      T     DBD    2210;


      CALL "GetValueR" (
           obj                      := 2874, // PointId = 019470, Station = PCU1
           rVal                     := #rVal);

      L     #rVal;
      T     DBD    2214;


      CALL "GetValueR" (
           obj                      := 2874, // PointId = 019470, Station = PCU1
           rVal                     := #rVal);

      L     #rVal;
      T     DBD    2218;


      CALL "GetValueR" (
           obj                      := 3023, // PointId = 029010, Station = PCU1
           rVal                     := #rVal);

      L     #rVal;
      T     DBD    2222;


      CALL "GetValueR" (
           obj                      := 3024, // PointId = 029020, Station = PCU1
           rVal                     := #rVal);

      L     #rVal;
      T     DBD    2226;


      CALL "GetValueR" (
           obj                      := 3025, // PointId = 029030, Station = PCU1
           rVal                     := #rVal);

      L     #rVal;
      T     DBD    2230;


      CALL "GetValueR" (
           obj                      := 3026, // PointId = 029040, Station = PCU1
           rVal                     := #rVal);

      L     #rVal;
      T     DBD    2234;


      CALL "GetValueR" (
           obj                      := 3027, // PointId = 029051, Station = PCU1
           rVal                     := #rVal);

      L     #rVal;
      T     DBD    2238;


      CALL "GetValueR" (
           obj                      := 3028, // PointId = 029060, Station = PCU1
           rVal                     := #rVal);

      L     #rVal;
      T     DBD    2242;


      CALL "GetValueR" (
           obj                      := 3029, // PointId = 029070, Station = PCU1
           rVal                     := #rVal);

      L     #rVal;
      T     DBD    2246;


      CALL "GetValueR" (
           obj                      := 3030, // PointId = 029080, Station = PCU1
           rVal                     := #rVal);

      L     #rVal;
      T     DBD    2250;


      CALL "GetValueR" (
           obj                      := 3031, // PointId = 029090, Station = PCU1
           rVal                     := #rVal);

      L     #rVal;
      T     DBD    2254;


      CALL "GetValueR" (
           obj                      := 3032, // PointId = 029120, Station = PCU1
           rVal                     := #rVal);

      L     #rVal;
      T     DBD    2258;


      CALL "GetValueR" (
           obj                      := 3033, // PointId = 029130, Station = PCU1
           rVal                     := #rVal);

      L     #rVal;
      T     DBD    2262;


      CALL "GetValueR" (
           obj                      := 3034, // PointId = 029140, Station = PCU1
           rVal                     := #rVal);

      L     #rVal;
      T     DBD    2266;


      CALL "GetValueR" (
           obj                      := 3035, // PointId = 029150, Station = PCU1
           rVal                     := #rVal);

      L     #rVal;
      T     DBD    2270;


      CALL "GetValueR" (
           obj                      := 3036, // PointId = 029160, Station = PCU1
           rVal                     := #rVal);

      L     #rVal;
      T     DBD    2274;


      CALL "GetValueR" (
           obj                      := 3036, // PointId = 029160, Station = PCU1
           rVal                     := #rVal);

      L     #rVal;
      T     DBD    2278;


      CALL "GetValueR" (
           obj                      := 3036, // PointId = 029160, Station = PCU1
           rVal                     := #rVal);

      L     #rVal;
      T     DBD    2282;


      CALL "GetValueI" (
           obj                      := 234, // PointId = 029100, Station = PCU1
           iVal                     := #iVal);

      L     #iVal;
      T     DBD    2286;


      CALL "GetValueI" (
           obj                      := 235, // PointId = 029110, Station = PCU1
           iVal                     := #iVal);

      L     #iVal;
      T     DBD    2290;


      CALL "GetValueI" (
           obj                      := 236, // PointId = 029190, Station = PCU1
           iVal                     := #iVal);

      L     #iVal;
      T     DBD    2294;


      CALL "GetValueI" (
           obj                      := 237, // PointId = 029200, Station = PCU1
           iVal                     := #iVal);

      L     #iVal;
      T     DBD    2298;


      CALL "GetValueI" (
           obj                      := 238, // PointId = 029210, Station = PCU1
           iVal                     := #iVal);

      L     #iVal;
      T     DBD    2302;


      CALL "GetValueI" (
           obj                      := 239, // PointId = 029240, Station = PCU1
           iVal                     := #iVal);

      L     #iVal;
      T     DBD    2306;


      CALL "GetValueI" (
           obj                      := 240, // PointId = 029260, Station = PCU1
           iVal                     := #iVal);

      L     #iVal;
      T     DBD    2310;


      CALL "GetValueI" (
           obj                      := 241, // PointId = 029270, Station = PCU1
           iVal                     := #iVal);

      L     #iVal;
      T     DBD    2314;


      CALL "GetValueI" (
           obj                      := 242, // PointId = 029290, Station = PCU1
           iVal                     := #iVal);

      L     #iVal;
      T     DBD    2318;


      CALL "GetValueI" (
           obj                      := 242, // PointId = 029290, Station = PCU1
           iVal                     := #iVal);

      L     #iVal;
      T     DBD    2322;


      CALL "GetValueR" (
           obj                      := 3038, // PointId = 029300, Station = PCU1
           rVal                     := #rVal);

      L     #rVal;
      T     DBD    2326;


      CALL "GetValueR" (
           obj                      := 2875, // PointId = 020051, Station = PCU1
           rVal                     := #rVal);

      L     #rVal;
      T     DBD    2330;


      CALL "GetValueR" (
           obj                      := 2876, // PointId = 020060, Station = PCU1
           rVal                     := #rVal);

      L     #rVal;
      T     DBD    2334;


      CALL "GetValueR" (
           obj                      := 2877, // PointId = 020070, Station = PCU1
           rVal                     := #rVal);

      L     #rVal;
      T     DBD    2338;


      CALL "GetValueR" (
           obj                      := 2878, // PointId = 020080, Station = PCU1
           rVal                     := #rVal);

      L     #rVal;
      T     DBD    2342;


      CALL "GetValueR" (
           obj                      := 2879, // PointId = 020090, Station = PCU1
           rVal                     := #rVal);

      L     #rVal;
      T     DBD    2346;


      CALL "GetValueR" (
           obj                      := 2880, // PointId = 020100, Station = PCU1
           rVal                     := #rVal);

      L     #rVal;
      T     DBD    2350;


      CALL "GetValueR" (
           obj                      := 3084, // PointId = 051170, Station = PCU1
           rVal                     := #rVal);

      L     #rVal;
      T     DBD    2354;


      CALL "GetValueR" (
           obj                      := 3085, // PointId = 051180, Station = PCU1
           rVal                     := #rVal);

      L     #rVal;
      T     DBD    2358;


      CALL "GetValueR" (
           obj                      := 3085, // PointId = 051180, Station = PCU1
           rVal                     := #rVal);

      L     #rVal;
      T     DBD    2362;


      CALL "GetValueI" (
           obj                      := 86, // PointId = 017650, Station = PCU1
           iVal                     := #iVal);

      L     #iVal;
      T     DBD    2366;


      CALL "GetValueI" (
           obj                      := 100, // PointId = 018650, Station = PCU1
           iVal                     := #iVal);

      L     #iVal;
      T     DBD    2370;


      CALL "GetValueI" (
           obj                      := 114, // PointId = 019650, Station = PCU1
           iVal                     := #iVal);

      L     #iVal;
      T     DBD    2374;

      BEA   ;
END_FUNCTION



DATA_BLOCK "abvspu_DB_DataLinkPLC"
TITLE = abvspu_DB_DataLinkPLC
AUTHOR : ab_de2zehr0
FAMILY : AbvSpu
NAME : DB_DLPLC
VERSION : 0.1


  STRUCT
   wCount : WORD  := W#16#252;	// Number of DWORD values
   adw : ARRAY  [0 .. 593 ] OF DWORD ;
  END_STRUCT ;
BEGIN
   wCount := W#16#252;
END_DATA_BLOCK

